(* Logix 5000 AddOnInstructionDefinition export Banner_QS18E_Param_v3; software revision 30.00 *)

TYPE Banner_IOL_Port_v2 :   // UDT that has all of the data items necessary to communicate with a specific Port on a IO-Link Master
STRUCT
   Port_Controlled : INT;   // Each bit represents a port on an IO-Link Master. Set to 1 to tell AOI to control that port.
   Port_Activate : INT;   // Each bit represents a port on an IO-Link Master. When ON that port will process any commands in queue.
   Port_Read : INT;   // Each bit represents a port on an IO-Link Master. Used to determine when device AOI has requested a Read command.
   Port_Write : INT;   // Each bit represents a port on an IO-Link Master. Used to determine when device AOI has requested a Write command.
   Port_RW_Complete : INT;   // Each bit represents a port on an IO-Link Master. Tells device AOI that Read or Write request has been completed.
   Port_Device_Read : INT;
   Data_Transfer : SINT[70];   // Array to transfer data from IO-Master to device AOIs.
END_STRUCT
END_TYPE

TYPE Banner_QS18E_1 :   // Parameters for D, DV, LP, CV, and FP type sensors.
STRUCT
   Response_Speed : SINT;   // 0 = High Speed, 1 = Standard, 2 = Robust.
   Polarity_of_Pins_2_and_4 : SINT;   // 0 = Push Pull, 1 = PNP, 2 = NPN.
   Pin_2_Config : SINT;   // 0 = Deactivated, 1 = Pin 2 Emitter Enable, 2 = Pin 2 Emitter Disable, 3 = Remote Input, 4 = Detection Output, 5 = Complimentary Output, 6 = Normally Closed Health, 7 = Normally Open Health, 8 = Normally Closed Marginal, 9 = Normally Open Marginal.
   Process_Data_Input_Config : SINT;   // 0 = 5 and Signal, 1 = 5 and Count, 2 = 5 and Duration, 3 = 5 and Events per Minute.
   Marginal_Mode : SINT;   // 0 = Marginal Disabled, 1 = Marginal Auto, 2 = Marginal User.
   User_Marginal_Light : INT;   // 0 to 1000. User defined threshold.
   User_Marginal_Dark : INT;   // 0 to 1000. User defined threshold.
   LED_Power : SINT;   // 0 = Auto, 1 = Min Power, 2 = Power 2, 3 = Power 3, 4 = Power 4, 5 = Power 5, 6 = Max Power.
END_STRUCT
END_TYPE

TYPE Banner_QS18E_2 :   // Parameters for EV and E type sensors
STRUCT
   Polarity_of_Pins_2_and_4 : SINT;   // 0 = Push Pull, 1 = PNP, 2 = NPN.
   Pin_2_Config : SINT;   // 0 = Deactivated, 1 = Pin 2 Emitter Enable, 2 = Pin 2 Emitter Disable, 3 = Remote Input, 4 = Detection Output, 5 = Complimentary Output, 6 = Normally Closed Health, 7 = Normally Open Health, 8 = Normally Closed Marginal, 9 = Normally Open Marginal.
   Frequency_Selection : SINT;   // 0 = High Speed, 1 = A, 2 = B, 3 = C.
   Power_Level : SINT;   // 0 to 5. Example: 5 = Power Level 5.
   Pushbutton_Lockout : SINT;   // 0 = Unlocked, 1 = Locked.
END_STRUCT
END_TYPE

TYPE Banner_QS18E_3 :   // Parameters for RV and R type sensors
STRUCT
   Polarity_of_Pins_2_and_4 : SINT;   // 0 = Push Pull, 1 = PNP, 2 = NPN.
   Pin_2_Config : SINT;   // 0 = Deactivated, 1 = Pin 2 Emitter Enable, 2 = Pin 2 Emitter Disable, 3 = Remote Input, 4 = Detection Output, 5 = Complimentary Output, 6 = Normally Closed Health, 7 = Normally Open Health, 8 = Normally Closed Marginal, 9 = Normally Open Marginal.
   Process_Data_Input_Config : SINT;   // 0 = 5 and Signal, 1 = 5 and Count, 2 = 5 and Duration, 3 = 5 and Events per Minute.
   Marginal_Mode : SINT;   // 0 = Marginal Disabled, 1 = Marginal Auto, 2 = Marginal User.
   User_Marginal_Light : INT;   // 0 to 1000. User defined threshold.
   User_Marginal_Dark : INT;   // 0 to 1000. User defined threshold.
   Frequency_Selection : SINT;   // 0 = High Speed, 1 = A, 2 = B, 3 = C.
   IOL_Filter_Time : INT;   // Time in ms to average IOL process data measurement between updates.
   Gain : SINT;   // 0 = Auto - Teach, 1 = Auto - Run, 2 = Low Gain, 3 = Mid Gain, 4 = High Gain.
   Pushbutton_Lockout : SINT;   // 0 = Unlocked, 1 = Locked.
END_STRUCT
END_TYPE

TYPE Banner_QS18E_RD_v3 :   // UDT that stores the Write Data for a QS18E.
STRUCT
   Master_Cycle_Time : INT;
   Min_Cycle_Time : INT;
   M_Sequence_Capability : INT;
   IO_Link_Version_ID : INT;
   Process_Data_Input_Length : INT;
   Process_Data_Output_Length : INT;
   Combined_Vendor_ID : DINT;   // IO-Link Vendor ID
   Vendor_ID1 : INT;
   Vendor_ID2 : INT;
   Combined_Device_ID : DINT;   // IO-Link Device ID
   Device_ID1 : INT;
   Device_ID2 : INT;
   Device_ID3 : INT;
   Serial_Number : STRING;
   All_Time_Run_Time : DINT;   // Read only counter that tracks the total time sensor has been running since manufacture. Value in Hours.
   Quality_of_Health : INT;
   Normalized_Signal_Strength : INT;
   Quality_of_Teach : INT;
   Health_Lower_Limit : INT;
   Health_Upper_Limit : INT;
   SP2_Lower_Sensing_Threshold : INT;
   SP2_Upper_Sensing_Threshold : INT;
   SP1_Lower_Sensing_Threshold : INT;
   SP1_Upper_Sensing_Threshold : INT;
   Sensor_Operationl_Mode : INT;
   Output_Event_Count : DINT;
   Output_Event_Duration : DINT;
   Output_Event_Frequency : DINT;
   Active_Margninal_Light_Threshold : DINT;
   Active_Marginal_Dark_Threshold : DINT;
   Sigal : DINT;   // Only available for Sensor Type 3. Raw ADC Signal value.
END_STRUCT
END_TYPE

TYPE Banner_QS18E_v3 :   // All of the parameters for a QS18E.
STRUCT
   Initial_Global_Read : BOOL;   // Determines if all of the IO-Link data has been read into the PLC yet
   Command : INT;   // Value placed in here will activate a read or write to a specifc IO-Link Index
   Read_Data : Banner_QS18E_RD_v3;   // Read Only Data
   Write_Data : Banner_QS18E_WD_v3;   // Write Data
   Archive : Banner_QS18E_WD_v3;   // Archive Data
   Reset : BOOL;   // Resets AOI. This will force a complete parameter read of the sensor.
END_STRUCT
END_TYPE

TYPE Banner_QS18E_WD_v3 :   // UDT that stores the Write Data for a QS18E.
STRUCT
   System_Command : INT;   // See IODD file for list of commands that can be activated via the System Command interface
   Parameter_Access_Lock : SINT;   // Write access to all parameters is prohibited while value is 1. Only this parameter can be adjusted when value is 1.
   Data_Storage_Lock : SINT;   // Automatic data storage is disabled when this value is equal to 1. Read access is not affected.
   Local_Parameterization_Lock : SINT;   // Parameterization via local control elements on device is disabled.
   Local_User_Interface_Lock : SINT;   // Operation of local user interface is disabled.
   BDC1_Swithpoint_Logic : INT;   // 0 = Light Operate, 1 = Dark Operate
   BDC1_BDC_Mode : INT;   // 1 = 1-Pt BGS, 128 = 2-Pt, 129 = Dynamic, 130 = Window or FGS, 131 = Dual
   BDC1_Hysteresis : DINT;   // Should always be 0
   Marginal_Signal_Delay : DINT;   // 0 to 60000. Millisecond value
   User_Health_Setting : INT;   // 0 to 90
   Offset_Percent : INT;   // 0 = Min, 1 = 10%, 2 = 15%, 3 = 20%, 4 = 25%, 5 = 30%, 6 = 40%, 7 = 50%, 8 = 100%, 9 = 200%.
   Auto_Compensaton : INT;   // 0=Disabled, 1=Enabled
   Delay_Timer_2 : DINT;   // 0 to 90000 ms
   Delay_Timer_1 : DINT;   // 0 to 90000 ms
   Delay_Mode : INT;   // 0=Disabled, 1=On Off Delay, 2=On One Shot, 3=Off One Shot
   Resettable_Run_Time : DINT;
   Type_1_Data : Banner_QS18E_1;   // Data for a D, DV, Lp, VC, or FP QS18E type sensor.
   Type_2_Data : Banner_QS18E_2;   // Data for a E or EV QS18E type sensor.
   Type_3_Data : Banner_QS18E_3;   // Data for a R or RV QS18E type sensor.
   All_Time_Run_Time_Event_Time : DINT;
   Resettable_Run_Time_Event_Time : DINT;
END_STRUCT
END_TYPE

ADD_ON_INSTRUCTION Banner_QS18E_Param_v3   (* revision 3.0, vendor Banner Engineering *)
// AOI to read and write parameter data to an IO-Link QS18E.
// Revision note:
// Updated for QS18 Emitter and Receiver.
VAR_IN_OUT
   QS18E : Banner_QS18E_v3; {required}
   Port_Data : Banner_IOL_Port_v2; {required}
END_VAR
VAR_INPUT
   Port : DINT; {required}
   Sensor_Type : DINT; {required}   // 1 = D, DV, LP, CV, & FP models, 2 = EV or E models, 3 = RV or R models.
END_VAR
VAR
   Local_Control : DINT; {access None}
   Global_Read_Command_Value : INT; {access None}
   Global_Write_Command_Value : INT; {access None}
   Command_Being_Processed : BOOL; {access None}
   Update_Archive : BOOL; {access None}
   Index_Write_Inprocess : INT; {access None}
   Index_Write_Control : INT; {access None}
   Inprocess_Index : DINT; {access None}
END_VAR

ROUTINE Logic   (* ladder *)
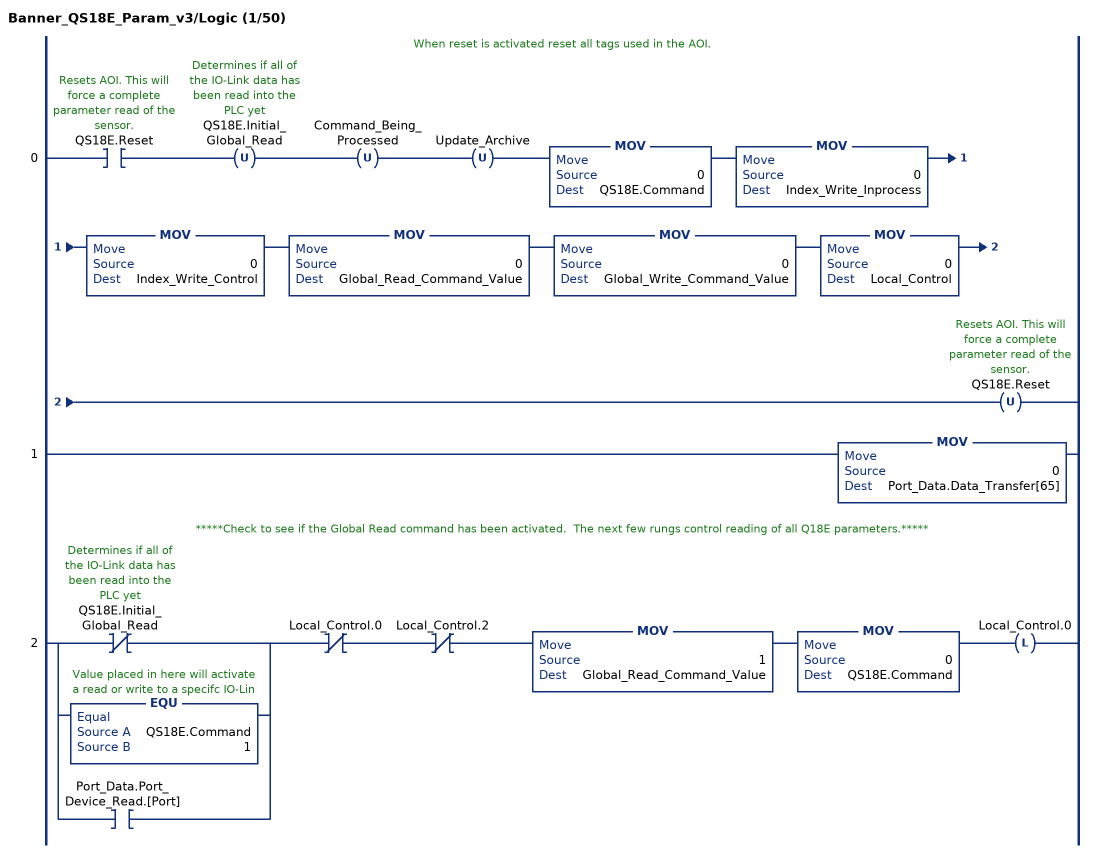
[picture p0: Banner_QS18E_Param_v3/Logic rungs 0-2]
   // When reset is activated reset all tags used in the AOI.
   0: XIC(QS18E.Reset)OTU(QS18E.Initial_Global_Read)OTU(Command_Being_Processed)OTU(Update_Archive)MOV(0,QS18E.Command)MOV(0,Index_Write_Inprocess)MOV(0,Index_Write_Control)MOV(0,Global_Read_Command_Value)MOV(0,Global_Write_Command_Value)MOV(0,Local_Control)OTU(QS18E.Reset);
   1: MOV(0,Port_Data.Data_Transfer[65]);
   // *****Check to see if the Global Read command has been activated.  The next few rungs control reading of all Q18E parameters.*****
   2: [XIO(QS18E.Initial_Global_Read) ,EQU(QS18E.Command,1) ,XIC(Port_Data.Port_Device_Read.[Port]) ]XIO(Local_Control.0)XIO(Local_Control.2)MOV(1,Global_Read_Command_Value)MOV(0,QS18E.Command)OTL(Local_Control.0);
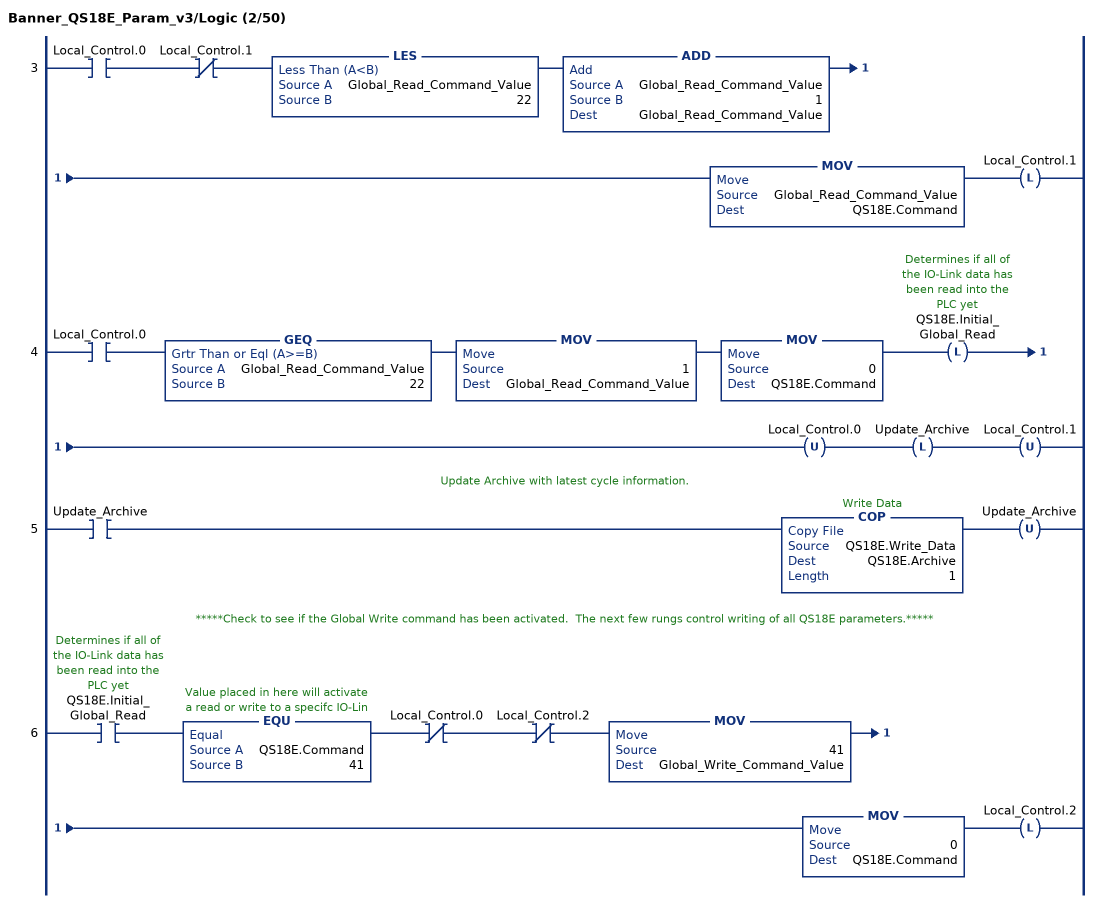
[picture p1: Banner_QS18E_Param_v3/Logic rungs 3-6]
   3: XIC(Local_Control.0)XIO(Local_Control.1)LES(Global_Read_Command_Value,22)ADD(Global_Read_Command_Value,1,Global_Read_Command_Value)MOV(Global_Read_Command_Value,QS18E.Command)OTL(Local_Control.1);
   4: XIC(Local_Control.0)GEQ(Global_Read_Command_Value,22)MOV(1,Global_Read_Command_Value)MOV(0,QS18E.Command)OTL(QS18E.Initial_Global_Read)OTU(Local_Control.0)OTL(Update_Archive)OTU(Local_Control.1);
   // Update Archive with latest cycle information.
   5: XIC(Update_Archive)COP(QS18E.Write_Data,QS18E.Archive,1)OTU(Update_Archive);
   // *****Check to see if the Global Write command has been activated.  The next few rungs control writing of all QS18E parameters.*****
   6: XIC(QS18E.Initial_Global_Read)EQU(QS18E.Command,41)XIO(Local_Control.0)XIO(Local_Control.2)MOV(41,Global_Write_Command_Value)MOV(0,QS18E.Command)OTL(Local_Control.2);
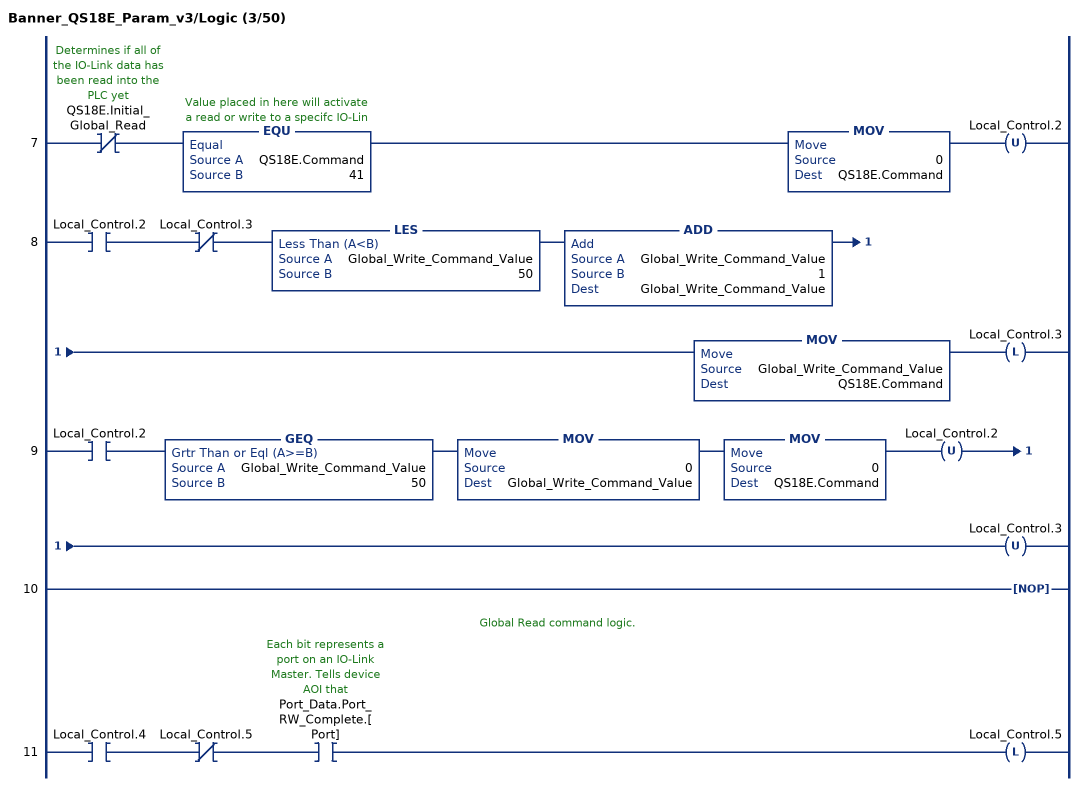
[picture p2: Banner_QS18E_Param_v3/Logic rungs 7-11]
   7: XIO(QS18E.Initial_Global_Read)EQU(QS18E.Command,41)MOV(0,QS18E.Command)OTU(Local_Control.2);
   8: XIC(Local_Control.2)XIO(Local_Control.3)LES(Global_Write_Command_Value,50)ADD(Global_Write_Command_Value,1,Global_Write_Command_Value)MOV(Global_Write_Command_Value,QS18E.Command)OTL(Local_Control.3);
   9: XIC(Local_Control.2)GEQ(Global_Write_Command_Value,50)MOV(0,Global_Write_Command_Value)MOV(0,QS18E.Command)OTU(Local_Control.2)OTU(Local_Control.3);
   10: NOP();
   // Global Read command logic.
   11: XIC(Local_Control.4)XIO(Local_Control.5)XIC(Port_Data.Port_RW_Complete.[Port])OTL(Local_Control.5);
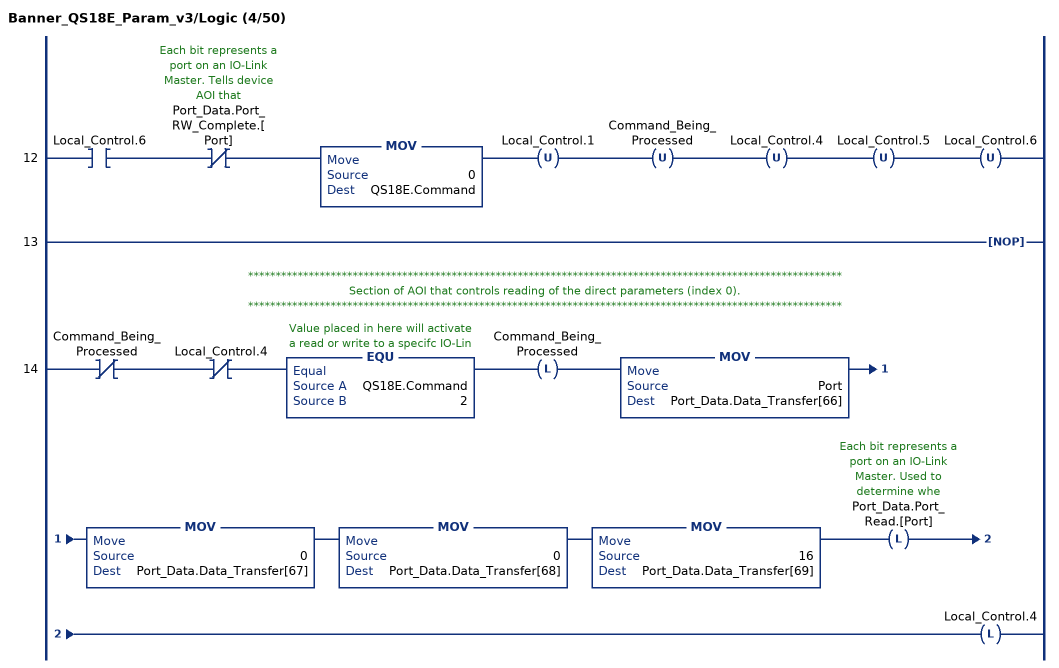
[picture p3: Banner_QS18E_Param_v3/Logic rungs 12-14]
   12: XIC(Local_Control.6)XIO(Port_Data.Port_RW_Complete.[Port])MOV(0,QS18E.Command)OTU(Local_Control.1)OTU(Command_Being_Processed)OTU(Local_Control.4)OTU(Local_Control.5)OTU(Local_Control.6);
   13: NOP();
   // ************************************************************************************************************
   // Section of AOI that controls reading of the direct parameters (index 0).
   // ************************************************************************************************************
   14: XIO(Command_Being_Processed)XIO(Local_Control.4)EQU(QS18E.Command,2)OTL(Command_Being_Processed)MOV(Port,Port_Data.Data_Transfer[66])MOV(0,Port_Data.Data_Transfer[67])MOV(0,Port_Data.Data_Transfer[68])MOV(16,Port_Data.Data_Transfer[69])OTL(Port_Data.Port_Read.[Port])OTL(Local_Control.4);
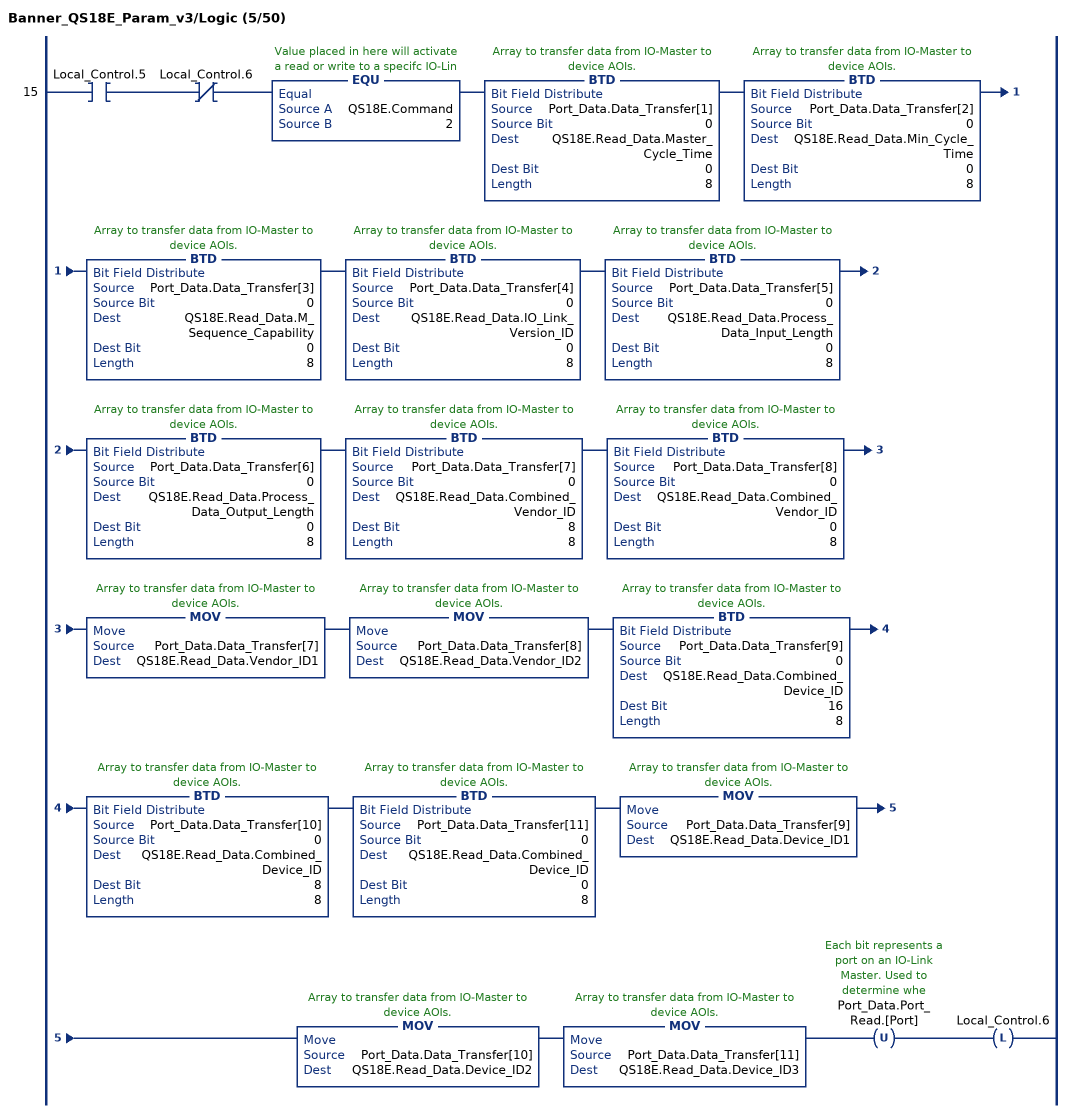
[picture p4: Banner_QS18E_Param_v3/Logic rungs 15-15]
   15: XIC(Local_Control.5)XIO(Local_Control.6)EQU(QS18E.Command,2)BTD(Port_Data.Data_Transfer[1],0,QS18E.Read_Data.Master_Cycle_Time,0,8)BTD(Port_Data.Data_Transfer[2],0,QS18E.Read_Data.Min_Cycle_Time,0,8)BTD(Port_Data.Data_Transfer[3],0,QS18E.Read_Data.M_Sequence_Capability,0,8)BTD(Port_Data.Data_Transfer[4],0,QS18E.Read_Data.IO_Link_Version_ID,0,8)BTD(Port_Data.Data_Transfer[5],0,QS18E.Read_Data.Process_Data_Input_Length,0,8)BTD(Port_Data.Data_Transfer[6],0,QS18E.Read_Data.Process_Data_Output_Length,0,8)BTD(Port_Data.Data_Transfer[7],0,QS18E.Read_Data.Combined_Vendor_ID,8,8)BTD(Port_Data.Data_Transfer[8],0,QS18E.Read_Data.Combined_Vendor_ID,0,8)MOV(Port_Data.Data_Transfer[7],QS18E.Read_Data.Vendor_ID1)MOV(Port_Data.Data_Transfer[8],QS18E.Read_Data.Vendor_ID2)BTD(Port_Data.Data_Transfer[9],0,QS18E.Read_Data.Combined_Device_ID,16,8)BTD(Port_Data.Data_Transfer[10],0,QS18E.Read_Data.Combined_Device_ID,8,8)BTD(Port_Data.Data_Transfer[11],0,QS18E.Read_Data.Combined_Device_ID,0,8)MOV(Port_Data.Data_Transfer[9],QS18E.Read_Data.Device_ID1)MOV(Port_Data.Data_Transfer[10],QS18E.Read_Data.Device_ID2)MOV(Port_Data.Data_Transfer[11],QS18E.Read_Data.Device_ID3)OTU(Port_Data.Port_Read.[Port])OTL(Local_Control.6);
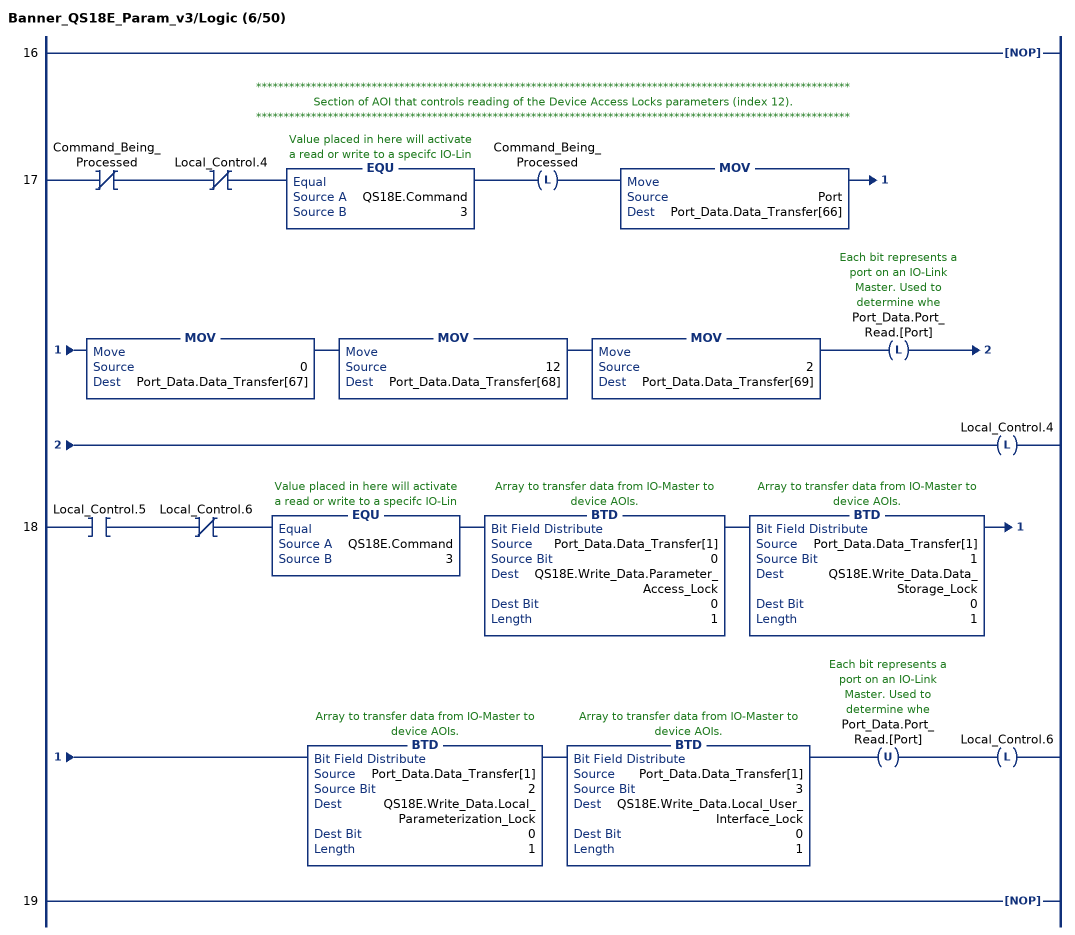
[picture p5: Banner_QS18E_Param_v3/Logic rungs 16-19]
   16: NOP();
   // ************************************************************************************************************
   // Section of AOI that controls reading of the Device Access Locks parameters (index 12).
   // ************************************************************************************************************
   17: XIO(Command_Being_Processed)XIO(Local_Control.4)EQU(QS18E.Command,3)OTL(Command_Being_Processed)MOV(Port,Port_Data.Data_Transfer[66])MOV(0,Port_Data.Data_Transfer[67])MOV(12,Port_Data.Data_Transfer[68])MOV(2,Port_Data.Data_Transfer[69])OTL(Port_Data.Port_Read.[Port])OTL(Local_Control.4);
   18: XIC(Local_Control.5)XIO(Local_Control.6)EQU(QS18E.Command,3)BTD(Port_Data.Data_Transfer[1],0,QS18E.Write_Data.Parameter_Access_Lock,0,1)BTD(Port_Data.Data_Transfer[1],1,QS18E.Write_Data.Data_Storage_Lock,0,1)BTD(Port_Data.Data_Transfer[1],2,QS18E.Write_Data.Local_Parameterization_Lock,0,1)BTD(Port_Data.Data_Transfer[1],3,QS18E.Write_Data.Local_User_Interface_Lock,0,1)OTU(Port_Data.Port_Read.[Port])OTL(Local_Control.6);
   19: NOP();
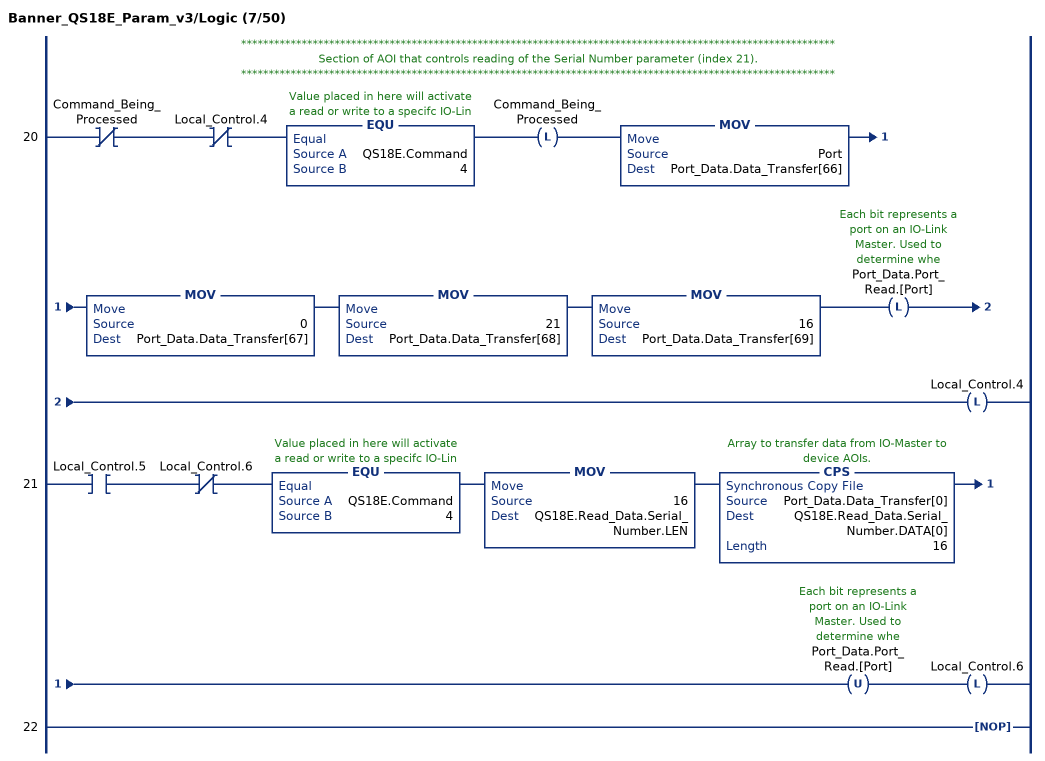
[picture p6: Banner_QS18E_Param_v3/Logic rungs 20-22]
   // ************************************************************************************************************
   // Section of AOI that controls reading of the Serial Number parameter (index 21).
   // ************************************************************************************************************
   20: XIO(Command_Being_Processed)XIO(Local_Control.4)EQU(QS18E.Command,4)OTL(Command_Being_Processed)MOV(Port,Port_Data.Data_Transfer[66])MOV(0,Port_Data.Data_Transfer[67])MOV(21,Port_Data.Data_Transfer[68])MOV(16,Port_Data.Data_Transfer[69])OTL(Port_Data.Port_Read.[Port])OTL(Local_Control.4);
   21: XIC(Local_Control.5)XIO(Local_Control.6)EQU(QS18E.Command,4)MOV(16,QS18E.Read_Data.Serial_Number.LEN)CPS(Port_Data.Data_Transfer[0],QS18E.Read_Data.Serial_Number.DATA[0],16)OTU(Port_Data.Port_Read.[Port])OTL(Local_Control.6);
   22: NOP();
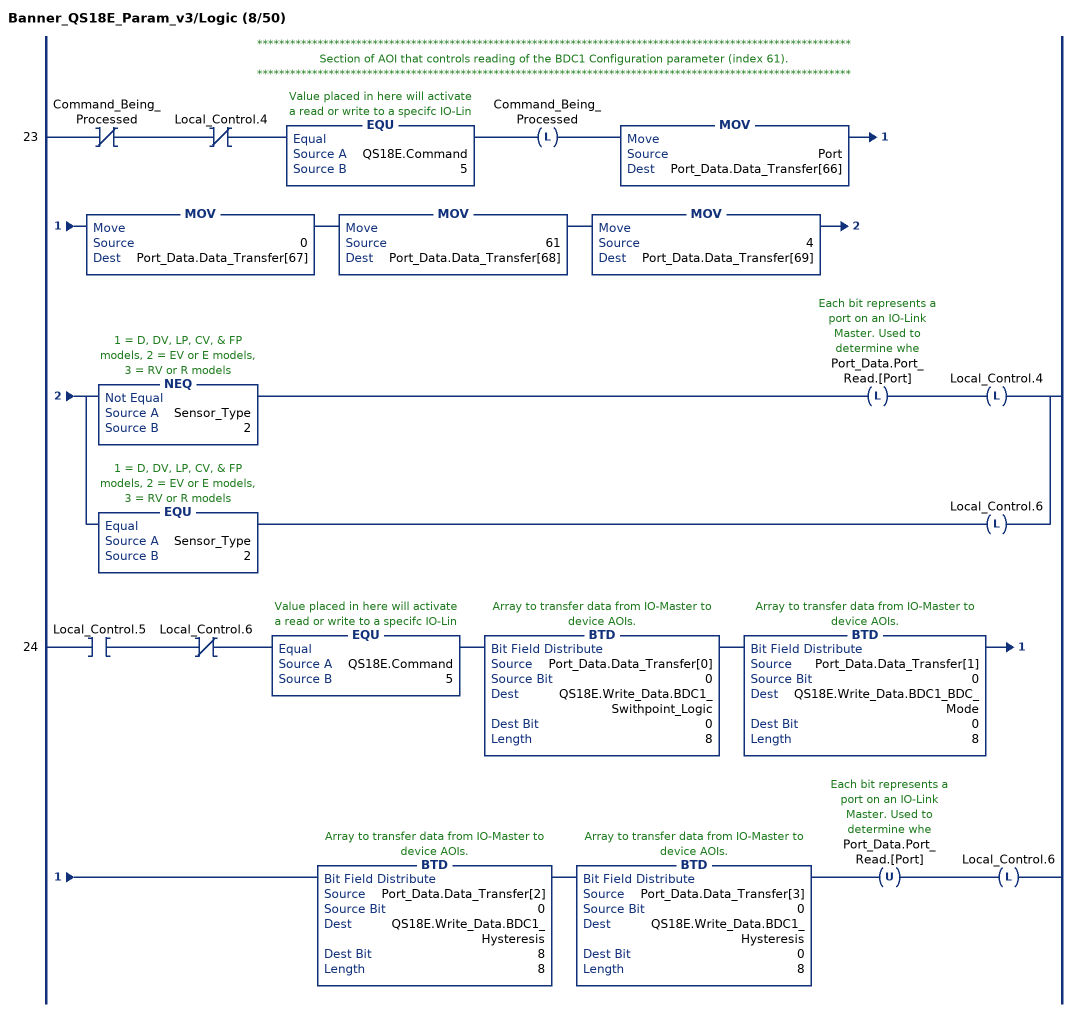
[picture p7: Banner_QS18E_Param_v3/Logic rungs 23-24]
   // ************************************************************************************************************
   // Section of AOI that controls reading of the BDC1 Configuration parameter (index 61).
   // ************************************************************************************************************
   23: XIO(Command_Being_Processed)XIO(Local_Control.4)EQU(QS18E.Command,5)OTL(Command_Being_Processed)MOV(Port,Port_Data.Data_Transfer[66])MOV(0,Port_Data.Data_Transfer[67])MOV(61,Port_Data.Data_Transfer[68])MOV(4,Port_Data.Data_Transfer[69])[NEQ(Sensor_Type,2) OTL(Port_Data.Port_Read.[Port]) OTL(Local_Control.4) ,EQU(Sensor_Type,2) OTL(Local_Control.6) ];
   24: XIC(Local_Control.5)XIO(Local_Control.6)EQU(QS18E.Command,5)BTD(Port_Data.Data_Transfer[0],0,QS18E.Write_Data.BDC1_Swithpoint_Logic,0,8)BTD(Port_Data.Data_Transfer[1],0,QS18E.Write_Data.BDC1_BDC_Mode,0,8)BTD(Port_Data.Data_Transfer[2],0,QS18E.Write_Data.BDC1_Hysteresis,8,8)BTD(Port_Data.Data_Transfer[3],0,QS18E.Write_Data.BDC1_Hysteresis,0,8)OTU(Port_Data.Port_Read.[Port])OTL(Local_Control.6);
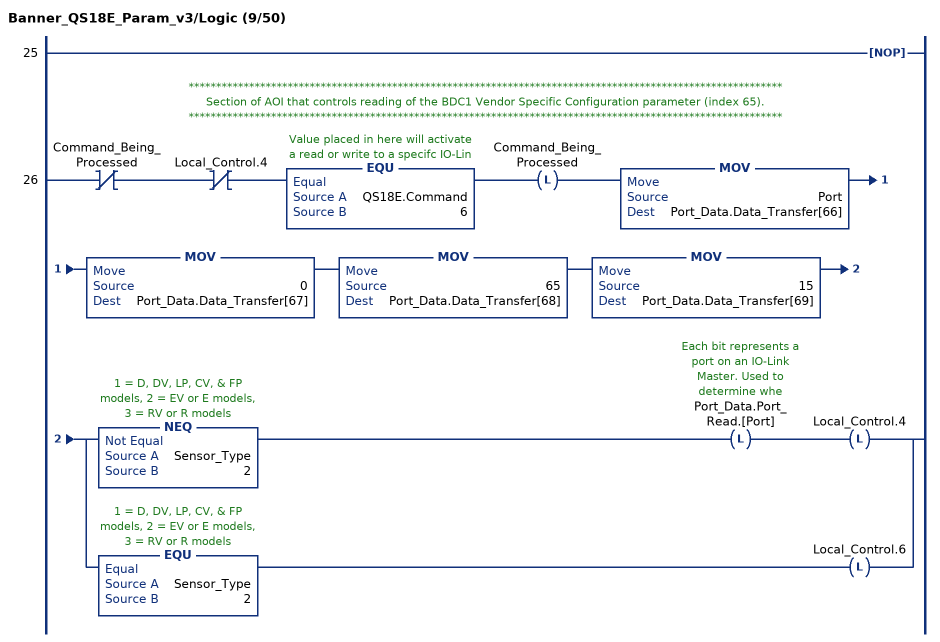
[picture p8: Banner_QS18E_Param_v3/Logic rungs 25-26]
   25: NOP();
   // ************************************************************************************************************
   // Section of AOI that controls reading of the BDC1 Vendor Specific Configuration parameter (index 65).
   // ************************************************************************************************************
   26: XIO(Command_Being_Processed)XIO(Local_Control.4)EQU(QS18E.Command,6)OTL(Command_Being_Processed)MOV(Port,Port_Data.Data_Transfer[66])MOV(0,Port_Data.Data_Transfer[67])MOV(65,Port_Data.Data_Transfer[68])MOV(15,Port_Data.Data_Transfer[69])[NEQ(Sensor_Type,2) OTL(Port_Data.Port_Read.[Port]) OTL(Local_Control.4) ,EQU(Sensor_Type,2) OTL(Local_Control.6) ];
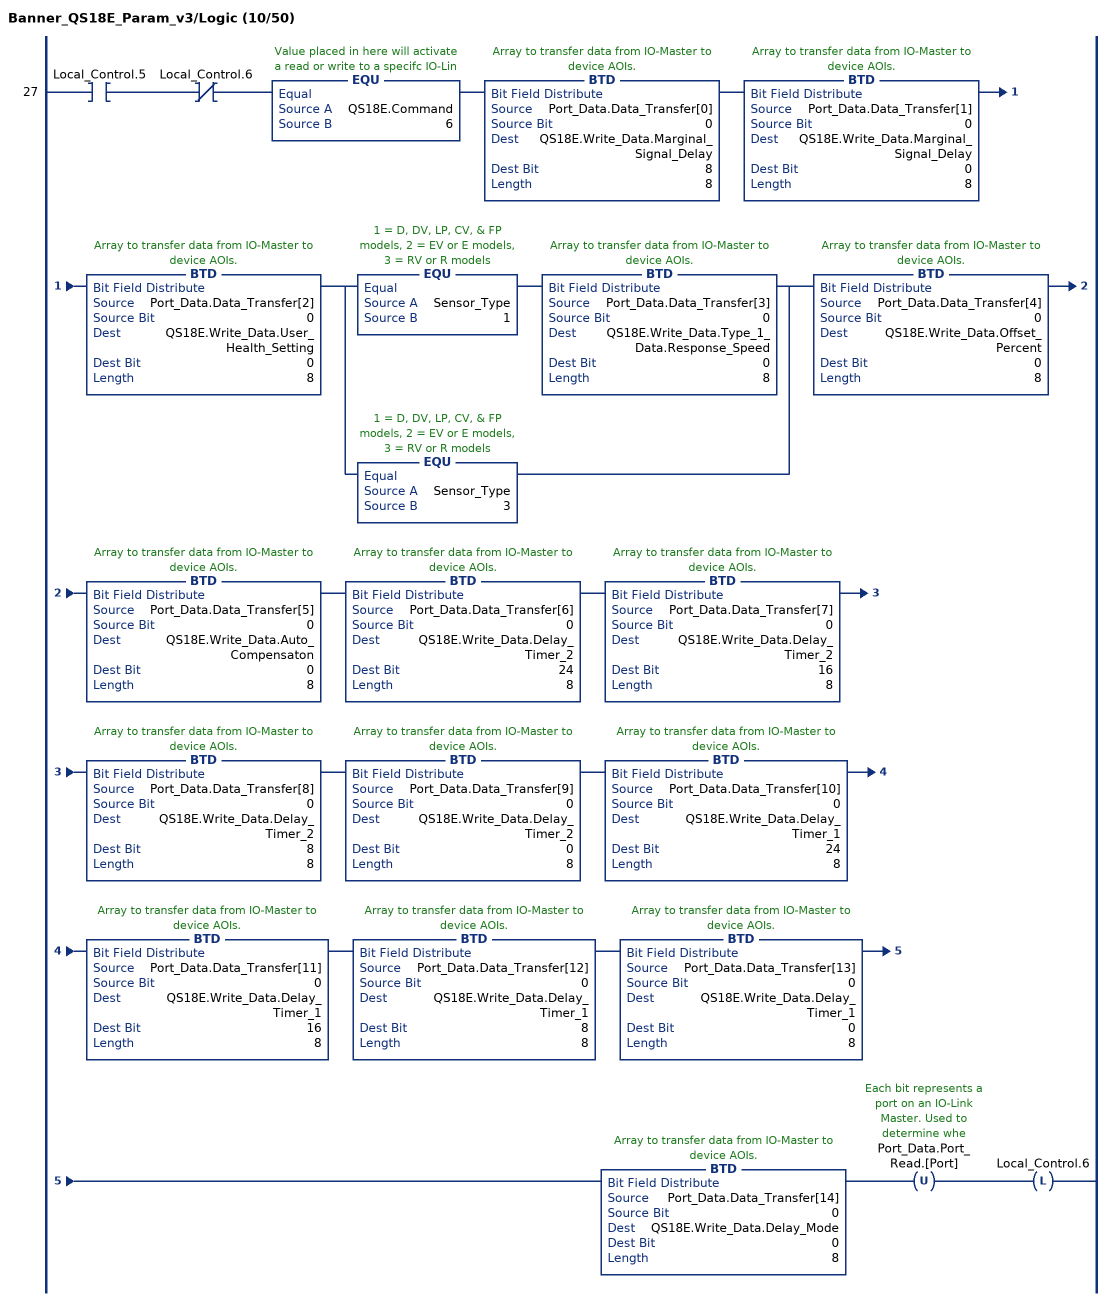
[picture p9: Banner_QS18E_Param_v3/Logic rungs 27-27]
   27: XIC(Local_Control.5)XIO(Local_Control.6)EQU(QS18E.Command,6)BTD(Port_Data.Data_Transfer[0],0,QS18E.Write_Data.Marginal_Signal_Delay,8,8)BTD(Port_Data.Data_Transfer[1],0,QS18E.Write_Data.Marginal_Signal_Delay,0,8)BTD(Port_Data.Data_Transfer[2],0,QS18E.Write_Data.User_Health_Setting,0,8)[EQU(Sensor_Type,1) BTD(Port_Data.Data_Transfer[3],0,QS18E.Write_Data.Type_1_Data.Response_Speed,0,8) ,EQU(Sensor_Type,3) ]BTD(Port_Data.Data_Transfer[4],0,QS18E.Write_Data.Offset_Percent,0,8)BTD(Port_Data.Data_Transfer[5],0,QS18E.Write_Data.Auto_Compensaton,0,8)BTD(Port_Data.Data_Transfer[6],0,QS18E.Write_Data.Delay_Timer_2,24,8)BTD(Port_Data.Data_Transfer[7],0,QS18E.Write_Data.Delay_Timer_2,16,8)BTD(Port_Data.Data_Transfer[8],0,QS18E.Write_Data.Delay_Timer_2,8,8)BTD(Port_Data.Data_Transfer[9],0,QS18E.Write_Data.Delay_Timer_2,0,8)BTD(Port_Data.Data_Transfer[10],0,QS18E.Write_Data.Delay_Timer_1,24,8)BTD(Port_Data.Data_Transfer[11],0,QS18E.Write_Data.Delay_Timer_1,16,8)BTD(Port_Data.Data_Transfer[12],0,QS18E.Write_Data.Delay_Timer_1,8,8)BTD(Port_Data.Data_Transfer[13],0,QS18E.Write_Data.Delay_Timer_1,0,8)BTD(Port_Data.Data_Transfer[14],0,QS18E.Write_Data.Delay_Mode,0,8)OTU(Port_Data.Port_Read.[Port])OTL(Local_Control.6);
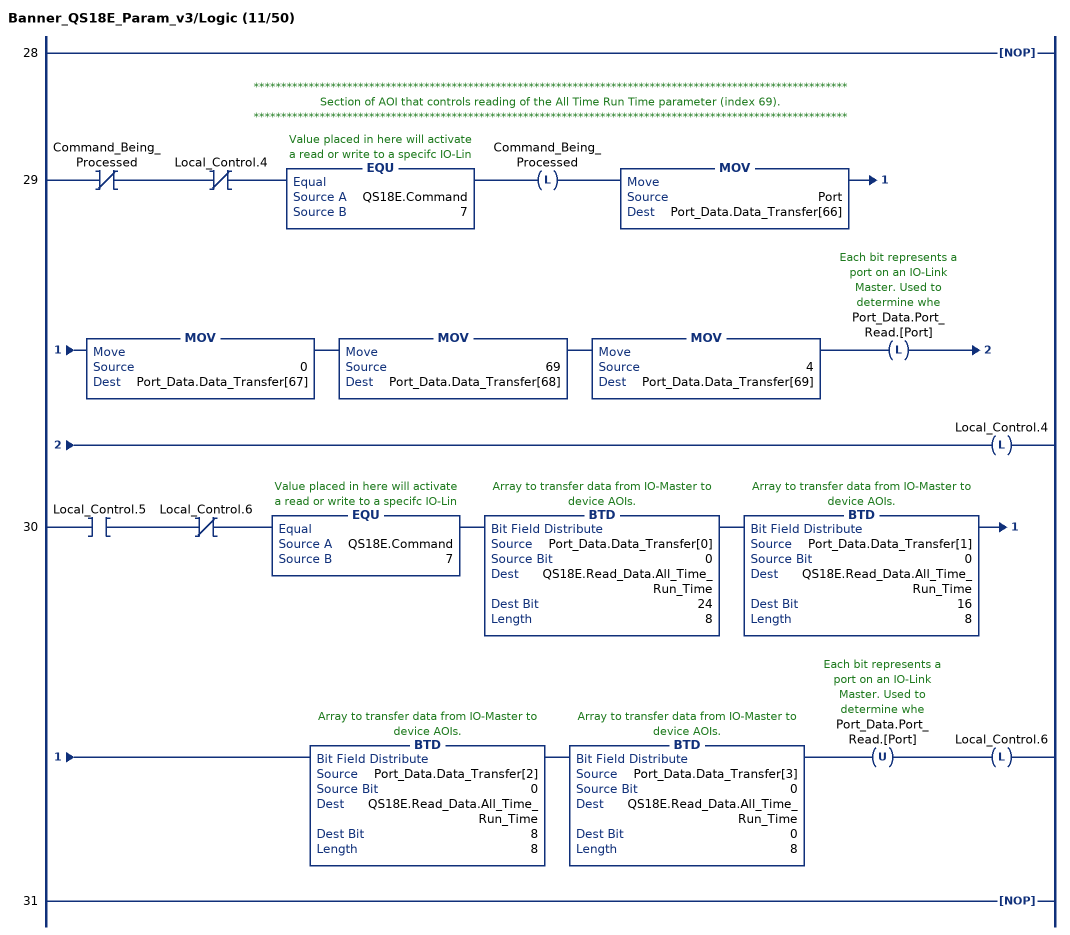
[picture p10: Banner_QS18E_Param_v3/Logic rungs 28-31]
   28: NOP();
   // ************************************************************************************************************
   // Section of AOI that controls reading of the All Time Run Time parameter (index 69).
   // ************************************************************************************************************
   29: XIO(Command_Being_Processed)XIO(Local_Control.4)EQU(QS18E.Command,7)OTL(Command_Being_Processed)MOV(Port,Port_Data.Data_Transfer[66])MOV(0,Port_Data.Data_Transfer[67])MOV(69,Port_Data.Data_Transfer[68])MOV(4,Port_Data.Data_Transfer[69])OTL(Port_Data.Port_Read.[Port])OTL(Local_Control.4);
   30: XIC(Local_Control.5)XIO(Local_Control.6)EQU(QS18E.Command,7)BTD(Port_Data.Data_Transfer[0],0,QS18E.Read_Data.All_Time_Run_Time,24,8)BTD(Port_Data.Data_Transfer[1],0,QS18E.Read_Data.All_Time_Run_Time,16,8)BTD(Port_Data.Data_Transfer[2],0,QS18E.Read_Data.All_Time_Run_Time,8,8)BTD(Port_Data.Data_Transfer[3],0,QS18E.Read_Data.All_Time_Run_Time,0,8)OTU(Port_Data.Port_Read.[Port])OTL(Local_Control.6);
   31: NOP();
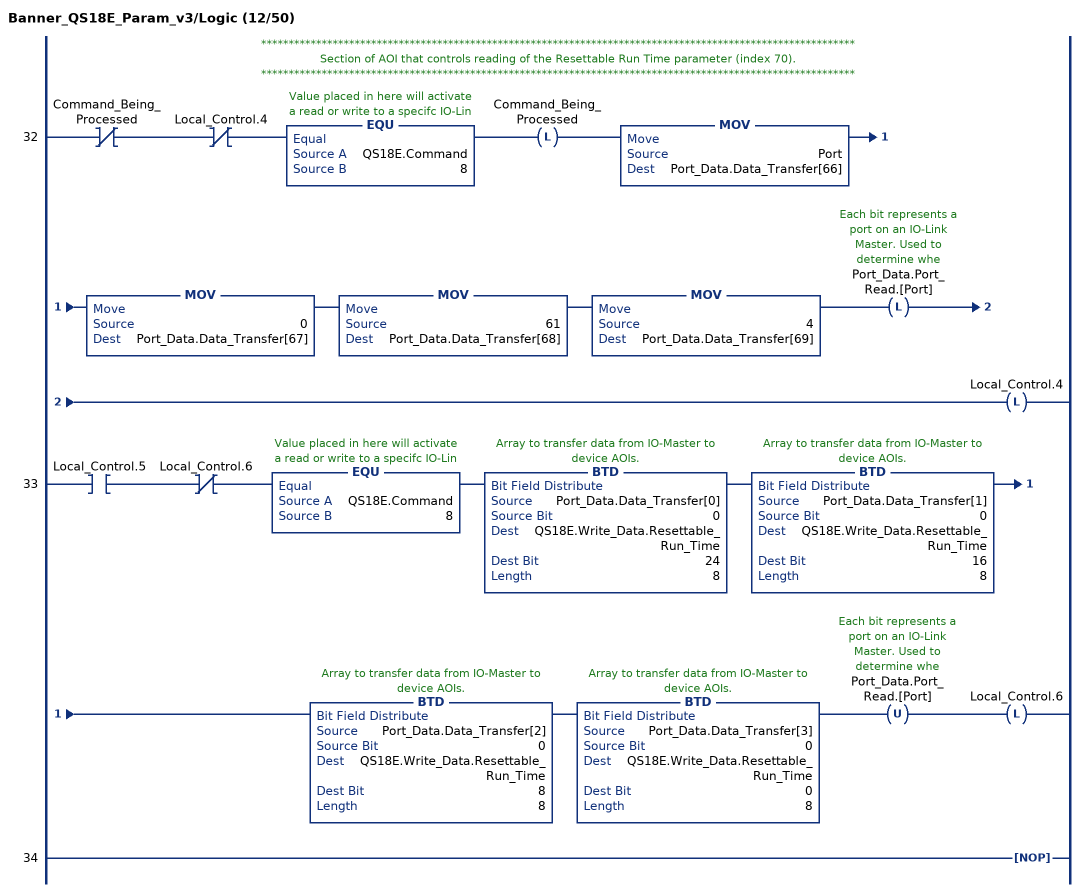
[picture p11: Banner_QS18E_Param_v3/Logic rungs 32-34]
   // ************************************************************************************************************
   // Section of AOI that controls reading of the Resettable Run Time parameter (index 70).
   // ************************************************************************************************************
   32: XIO(Command_Being_Processed)XIO(Local_Control.4)EQU(QS18E.Command,8)OTL(Command_Being_Processed)MOV(Port,Port_Data.Data_Transfer[66])MOV(0,Port_Data.Data_Transfer[67])MOV(61,Port_Data.Data_Transfer[68])MOV(4,Port_Data.Data_Transfer[69])OTL(Port_Data.Port_Read.[Port])OTL(Local_Control.4);
   33: XIC(Local_Control.5)XIO(Local_Control.6)EQU(QS18E.Command,8)BTD(Port_Data.Data_Transfer[0],0,QS18E.Write_Data.Resettable_Run_Time,24,8)BTD(Port_Data.Data_Transfer[1],0,QS18E.Write_Data.Resettable_Run_Time,16,8)BTD(Port_Data.Data_Transfer[2],0,QS18E.Write_Data.Resettable_Run_Time,8,8)BTD(Port_Data.Data_Transfer[3],0,QS18E.Write_Data.Resettable_Run_Time,0,8)OTU(Port_Data.Port_Read.[Port])OTL(Local_Control.6);
   34: NOP();
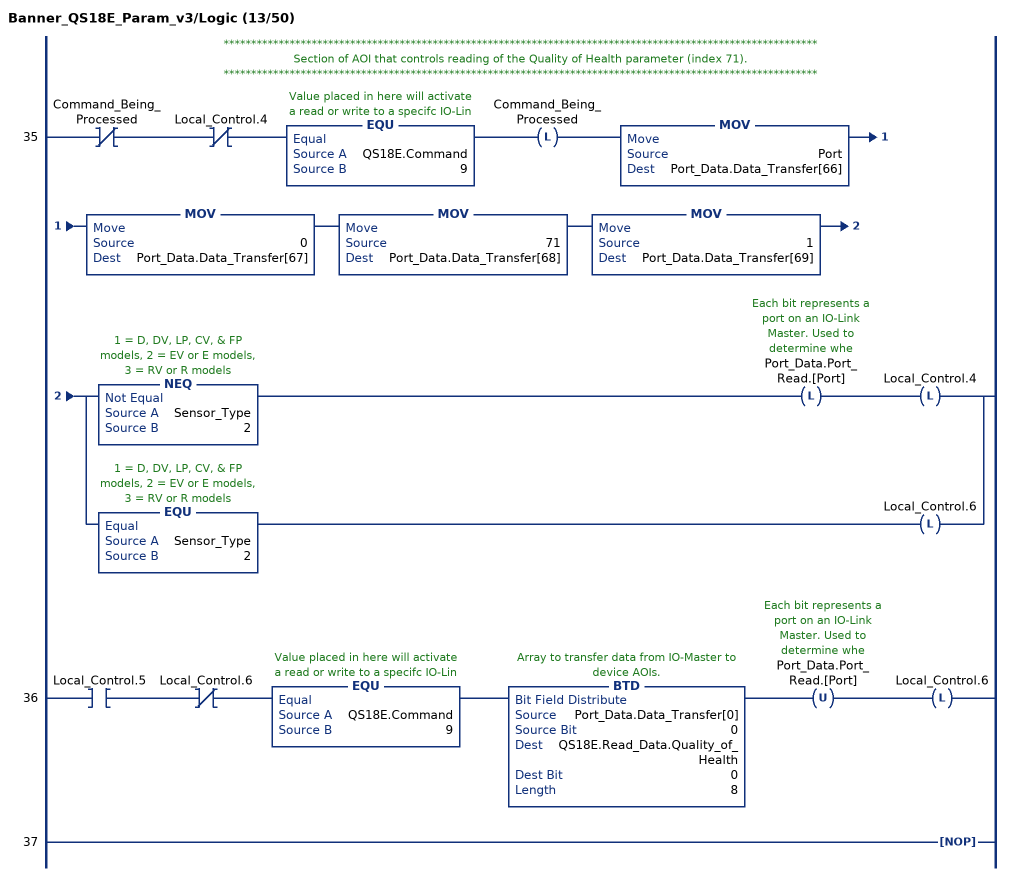
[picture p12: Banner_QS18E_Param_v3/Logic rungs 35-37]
   // ************************************************************************************************************
   // Section of AOI that controls reading of the Quality of Health parameter (index 71).
   // ************************************************************************************************************
   35: XIO(Command_Being_Processed)XIO(Local_Control.4)EQU(QS18E.Command,9)OTL(Command_Being_Processed)MOV(Port,Port_Data.Data_Transfer[66])MOV(0,Port_Data.Data_Transfer[67])MOV(71,Port_Data.Data_Transfer[68])MOV(1,Port_Data.Data_Transfer[69])[NEQ(Sensor_Type,2) OTL(Port_Data.Port_Read.[Port]) OTL(Local_Control.4) ,EQU(Sensor_Type,2) OTL(Local_Control.6) ];
   36: XIC(Local_Control.5)XIO(Local_Control.6)EQU(QS18E.Command,9)BTD(Port_Data.Data_Transfer[0],0,QS18E.Read_Data.Quality_of_Health,0,8)OTU(Port_Data.Port_Read.[Port])OTL(Local_Control.6);
   37: NOP();
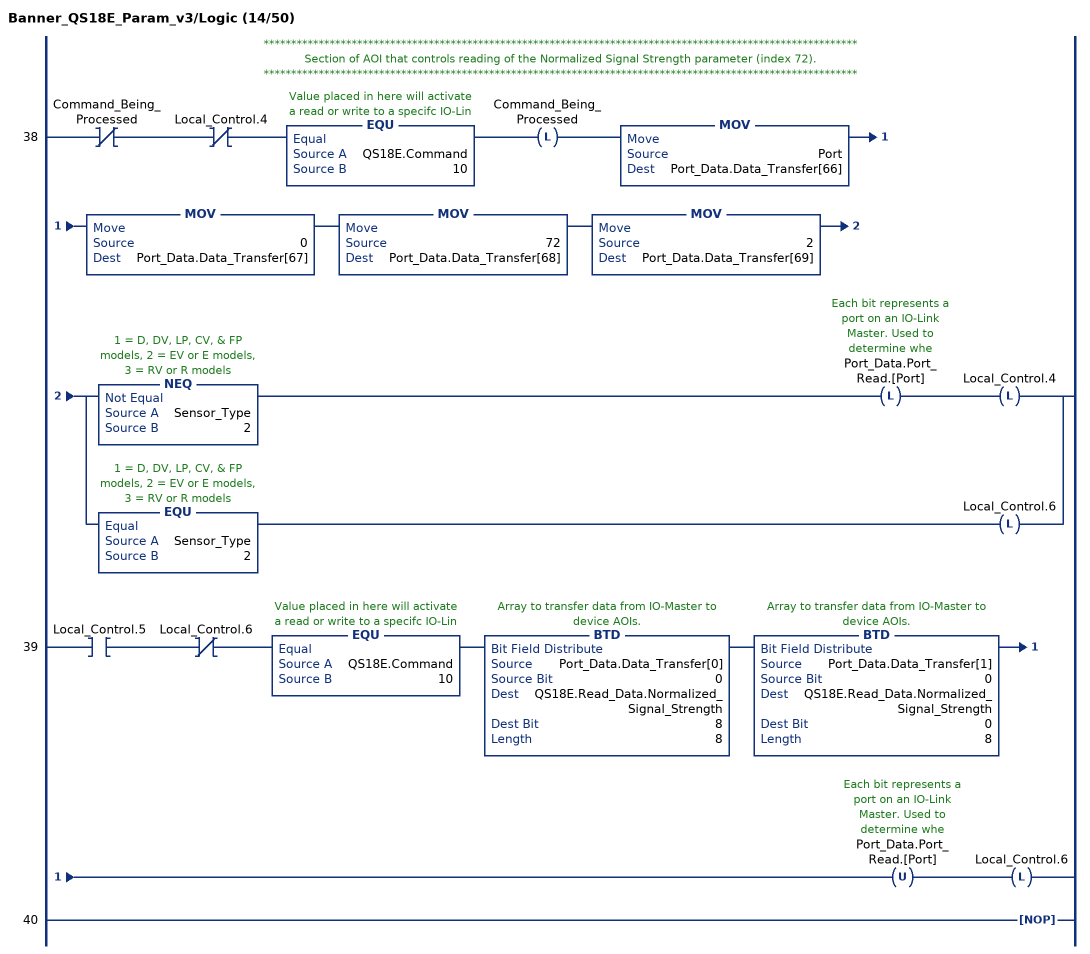
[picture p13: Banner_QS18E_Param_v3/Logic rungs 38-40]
   // ************************************************************************************************************
   // Section of AOI that controls reading of the Normalized Signal Strength parameter (index 72).
   // ************************************************************************************************************
   38: XIO(Command_Being_Processed)XIO(Local_Control.4)EQU(QS18E.Command,10)OTL(Command_Being_Processed)MOV(Port,Port_Data.Data_Transfer[66])MOV(0,Port_Data.Data_Transfer[67])MOV(72,Port_Data.Data_Transfer[68])MOV(2,Port_Data.Data_Transfer[69])[NEQ(Sensor_Type,2) OTL(Port_Data.Port_Read.[Port]) OTL(Local_Control.4) ,EQU(Sensor_Type,2) OTL(Local_Control.6) ];
   39: XIC(Local_Control.5)XIO(Local_Control.6)EQU(QS18E.Command,10)BTD(Port_Data.Data_Transfer[0],0,QS18E.Read_Data.Normalized_Signal_Strength,8,8)BTD(Port_Data.Data_Transfer[1],0,QS18E.Read_Data.Normalized_Signal_Strength,0,8)OTU(Port_Data.Port_Read.[Port])OTL(Local_Control.6);
   40: NOP();
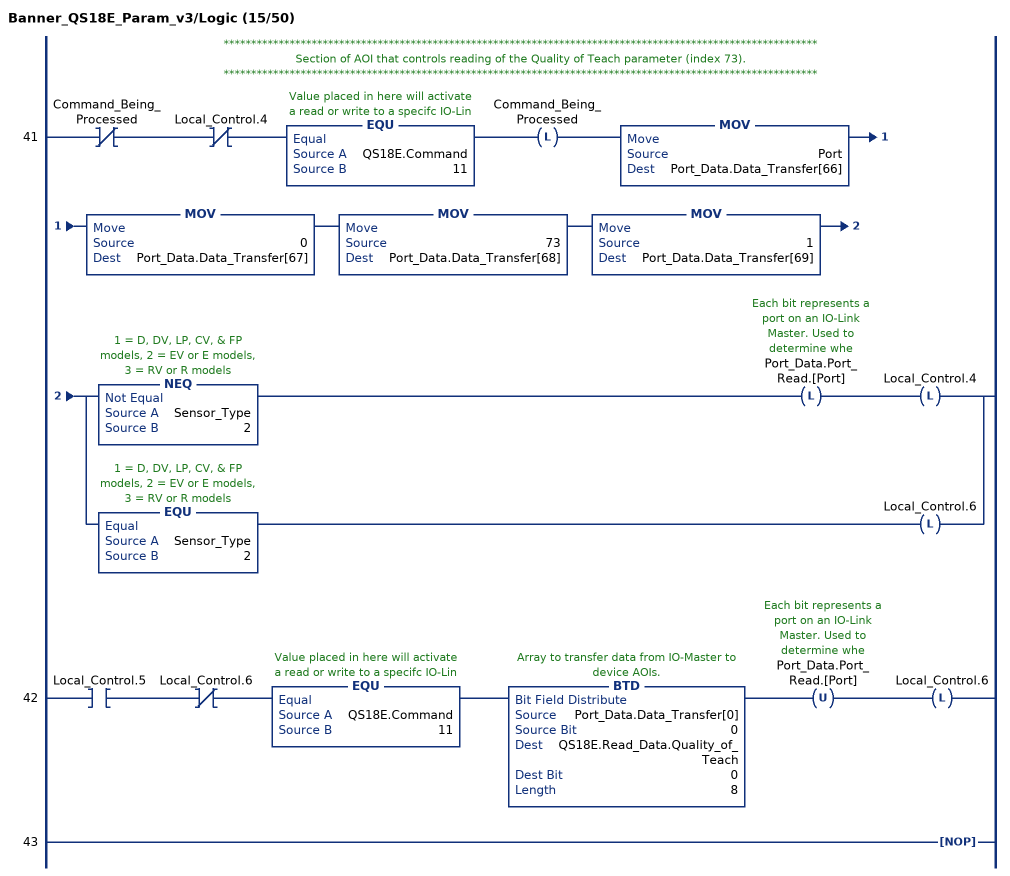
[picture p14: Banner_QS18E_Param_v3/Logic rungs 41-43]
   // ************************************************************************************************************
   // Section of AOI that controls reading of the Quality of Teach parameter (index 73).
   // ************************************************************************************************************
   41: XIO(Command_Being_Processed)XIO(Local_Control.4)EQU(QS18E.Command,11)OTL(Command_Being_Processed)MOV(Port,Port_Data.Data_Transfer[66])MOV(0,Port_Data.Data_Transfer[67])MOV(73,Port_Data.Data_Transfer[68])MOV(1,Port_Data.Data_Transfer[69])[NEQ(Sensor_Type,2) OTL(Port_Data.Port_Read.[Port]) OTL(Local_Control.4) ,EQU(Sensor_Type,2) OTL(Local_Control.6) ];
   42: XIC(Local_Control.5)XIO(Local_Control.6)EQU(QS18E.Command,11)BTD(Port_Data.Data_Transfer[0],0,QS18E.Read_Data.Quality_of_Teach,0,8)OTU(Port_Data.Port_Read.[Port])OTL(Local_Control.6);
   43: NOP();
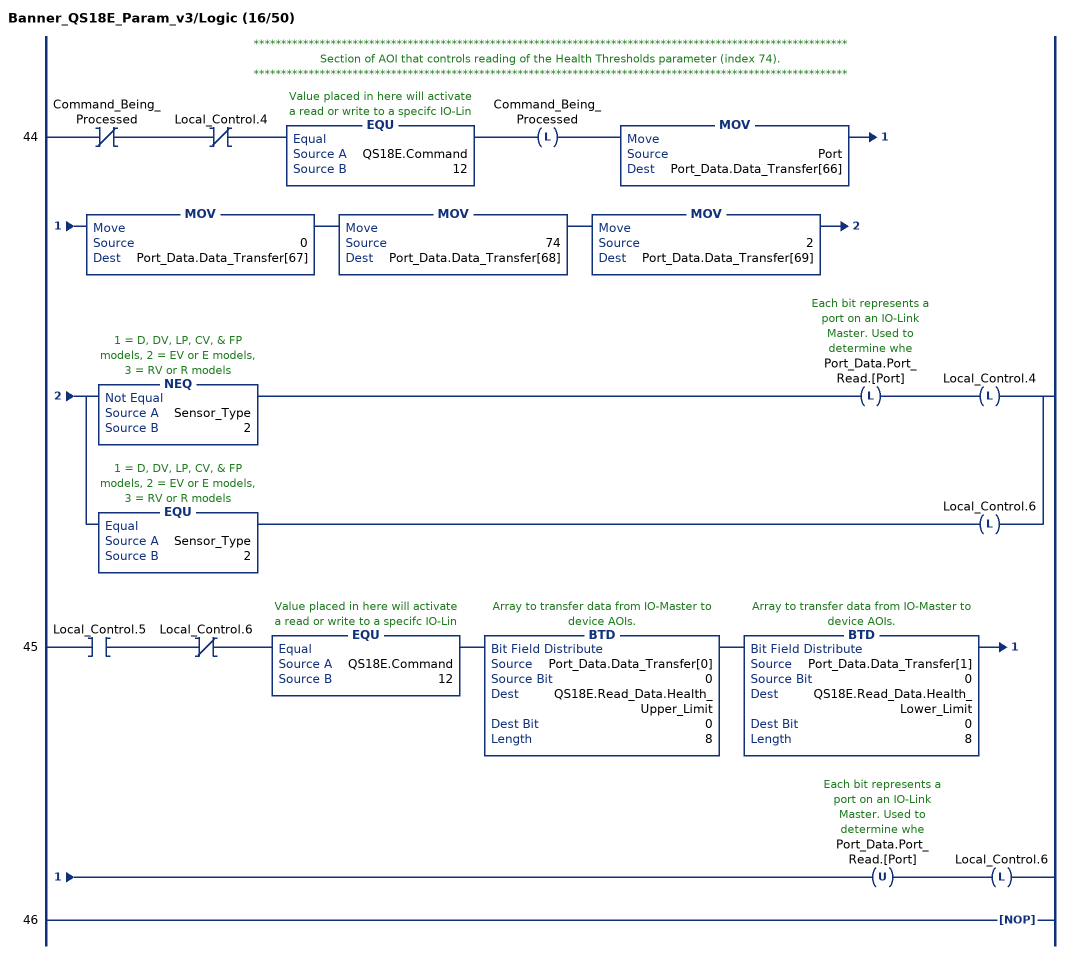
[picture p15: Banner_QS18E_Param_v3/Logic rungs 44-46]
   // ************************************************************************************************************
   // Section of AOI that controls reading of the Health Thresholds parameter (index 74).
   // ************************************************************************************************************
   44: XIO(Command_Being_Processed)XIO(Local_Control.4)EQU(QS18E.Command,12)OTL(Command_Being_Processed)MOV(Port,Port_Data.Data_Transfer[66])MOV(0,Port_Data.Data_Transfer[67])MOV(74,Port_Data.Data_Transfer[68])MOV(2,Port_Data.Data_Transfer[69])[NEQ(Sensor_Type,2) OTL(Port_Data.Port_Read.[Port]) OTL(Local_Control.4) ,EQU(Sensor_Type,2) OTL(Local_Control.6) ];
   45: XIC(Local_Control.5)XIO(Local_Control.6)EQU(QS18E.Command,12)BTD(Port_Data.Data_Transfer[0],0,QS18E.Read_Data.Health_Upper_Limit,0,8)BTD(Port_Data.Data_Transfer[1],0,QS18E.Read_Data.Health_Lower_Limit,0,8)OTU(Port_Data.Port_Read.[Port])OTL(Local_Control.6);
   46: NOP();
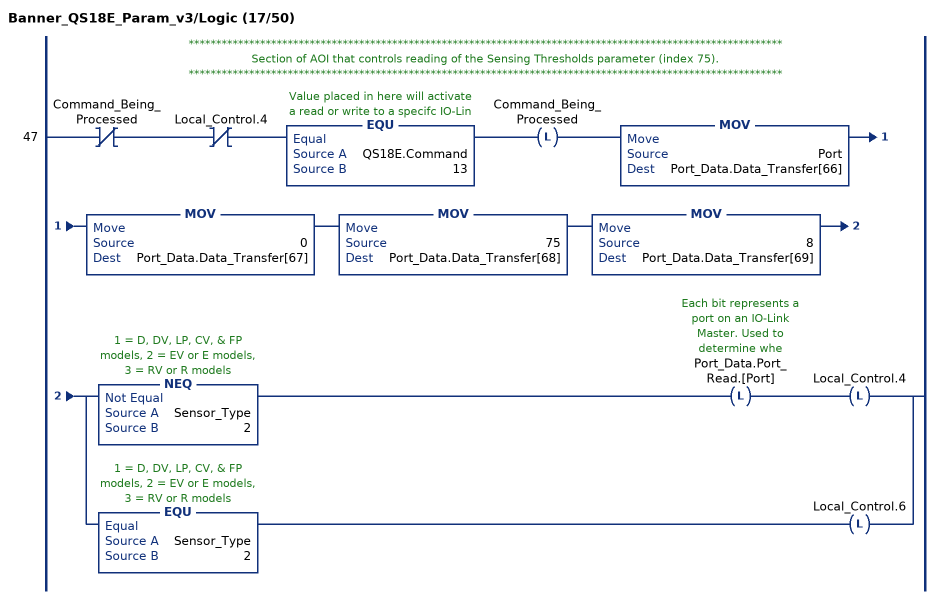
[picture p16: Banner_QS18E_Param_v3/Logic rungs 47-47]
   // ************************************************************************************************************
   // Section of AOI that controls reading of the Sensing Thresholds parameter (index 75).
   // ************************************************************************************************************
   47: XIO(Command_Being_Processed)XIO(Local_Control.4)EQU(QS18E.Command,13)OTL(Command_Being_Processed)MOV(Port,Port_Data.Data_Transfer[66])MOV(0,Port_Data.Data_Transfer[67])MOV(75,Port_Data.Data_Transfer[68])MOV(8,Port_Data.Data_Transfer[69])[NEQ(Sensor_Type,2) OTL(Port_Data.Port_Read.[Port]) OTL(Local_Control.4) ,EQU(Sensor_Type,2) OTL(Local_Control.6) ];
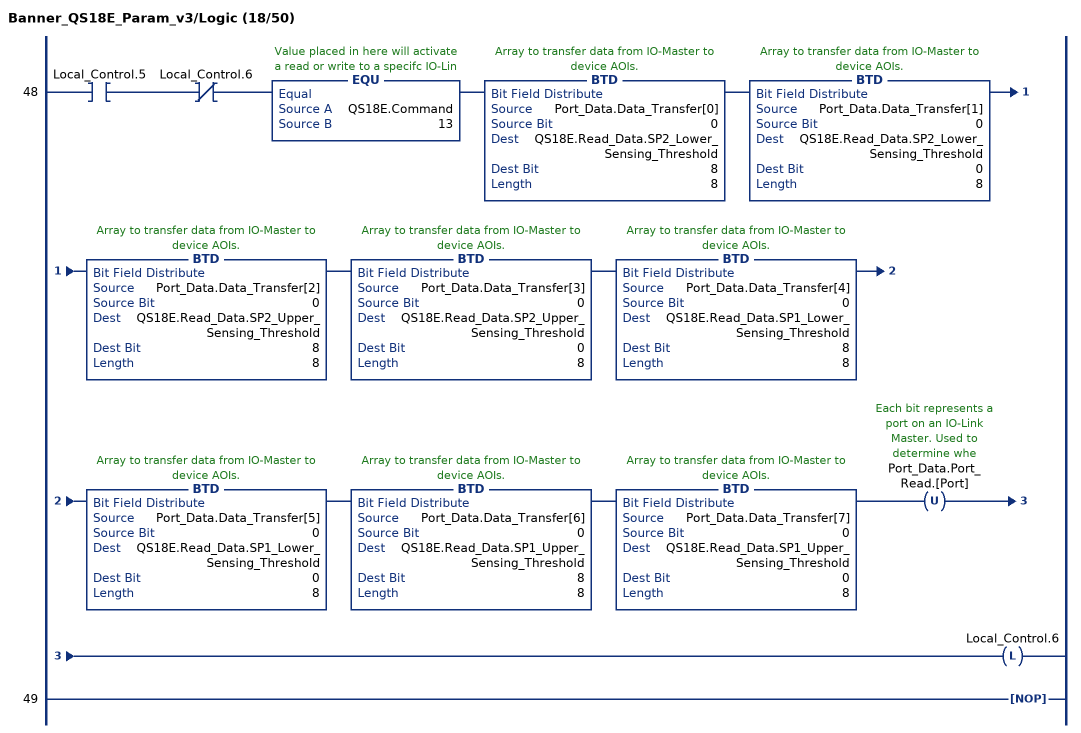
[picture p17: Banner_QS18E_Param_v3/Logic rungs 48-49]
   48: XIC(Local_Control.5)XIO(Local_Control.6)EQU(QS18E.Command,13)BTD(Port_Data.Data_Transfer[0],0,QS18E.Read_Data.SP2_Lower_Sensing_Threshold,8,8)BTD(Port_Data.Data_Transfer[1],0,QS18E.Read_Data.SP2_Lower_Sensing_Threshold,0,8)BTD(Port_Data.Data_Transfer[2],0,QS18E.Read_Data.SP2_Upper_Sensing_Threshold,8,8)BTD(Port_Data.Data_Transfer[3],0,QS18E.Read_Data.SP2_Upper_Sensing_Threshold,0,8)BTD(Port_Data.Data_Transfer[4],0,QS18E.Read_Data.SP1_Lower_Sensing_Threshold,8,8)BTD(Port_Data.Data_Transfer[5],0,QS18E.Read_Data.SP1_Lower_Sensing_Threshold,0,8)BTD(Port_Data.Data_Transfer[6],0,QS18E.Read_Data.SP1_Upper_Sensing_Threshold,8,8)BTD(Port_Data.Data_Transfer[7],0,QS18E.Read_Data.SP1_Upper_Sensing_Threshold,0,8)OTU(Port_Data.Port_Read.[Port])OTL(Local_Control.6);
   49: NOP();
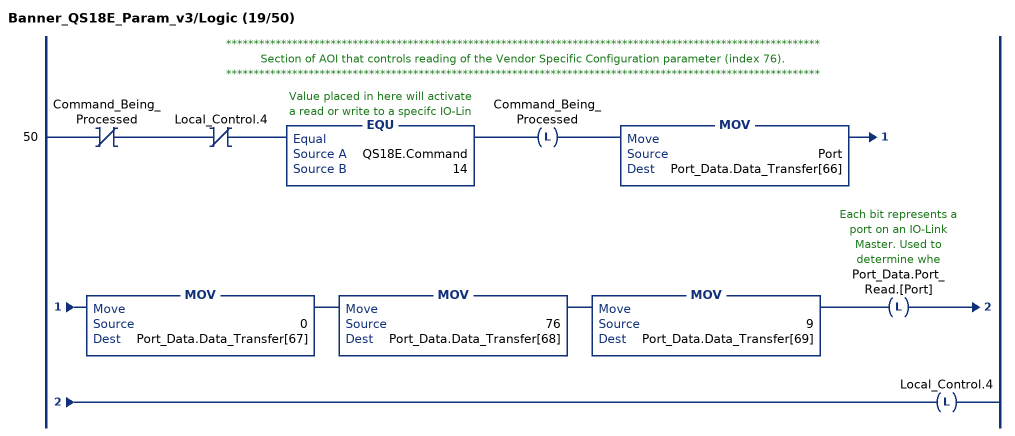
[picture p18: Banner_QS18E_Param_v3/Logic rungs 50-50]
   // ************************************************************************************************************
   // Section of AOI that controls reading of the Vendor Specific Configuration parameter (index 76).
   // ************************************************************************************************************
   50: XIO(Command_Being_Processed)XIO(Local_Control.4)EQU(QS18E.Command,14)OTL(Command_Being_Processed)MOV(Port,Port_Data.Data_Transfer[66])MOV(0,Port_Data.Data_Transfer[67])MOV(76,Port_Data.Data_Transfer[68])MOV(9,Port_Data.Data_Transfer[69])OTL(Port_Data.Port_Read.[Port])OTL(Local_Control.4);
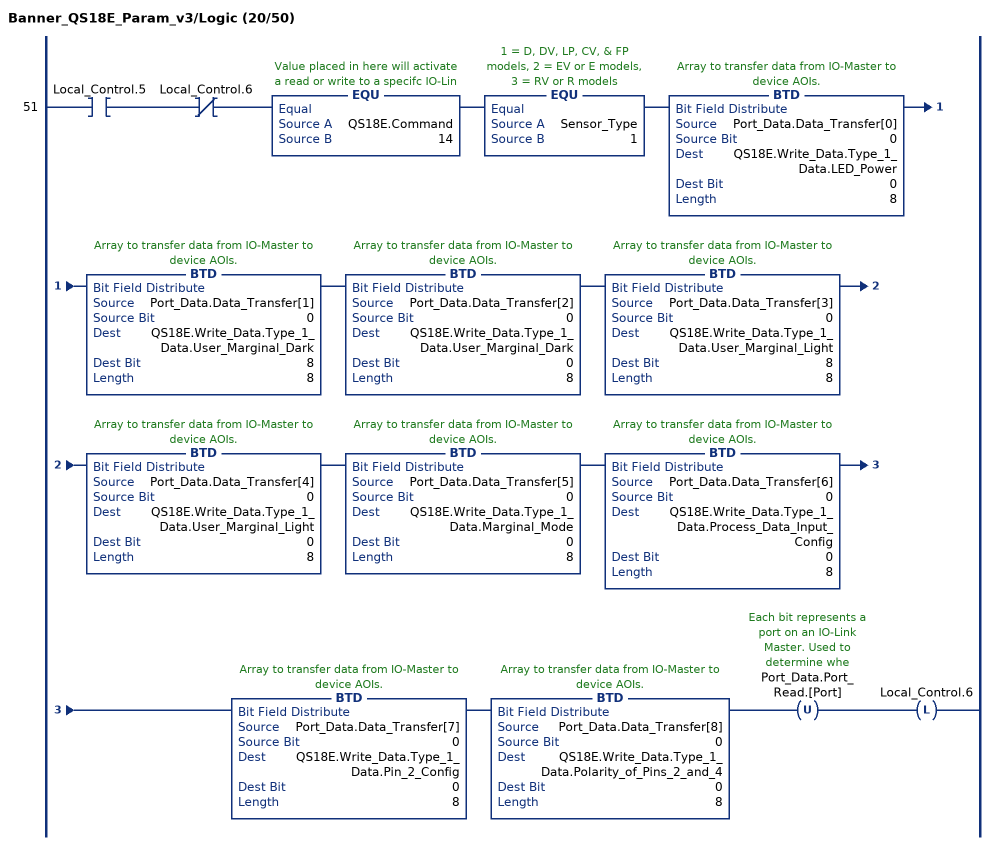
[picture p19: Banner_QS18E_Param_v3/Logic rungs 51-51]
   51: XIC(Local_Control.5)XIO(Local_Control.6)EQU(QS18E.Command,14)EQU(Sensor_Type,1)BTD(Port_Data.Data_Transfer[0],0,QS18E.Write_Data.Type_1_Data.LED_Power,0,8)BTD(Port_Data.Data_Transfer[1],0,QS18E.Write_Data.Type_1_Data.User_Marginal_Dark,8,8)BTD(Port_Data.Data_Transfer[2],0,QS18E.Write_Data.Type_1_Data.User_Marginal_Dark,0,8)BTD(Port_Data.Data_Transfer[3],0,QS18E.Write_Data.Type_1_Data.User_Marginal_Light,8,8)BTD(Port_Data.Data_Transfer[4],0,QS18E.Write_Data.Type_1_Data.User_Marginal_Light,0,8)BTD(Port_Data.Data_Transfer[5],0,QS18E.Write_Data.Type_1_Data.Marginal_Mode,0,8)BTD(Port_Data.Data_Transfer[6],0,QS18E.Write_Data.Type_1_Data.Process_Data_Input_Config,0,8)BTD(Port_Data.Data_Transfer[7],0,QS18E.Write_Data.Type_1_Data.Pin_2_Config,0,8)BTD(Port_Data.Data_Transfer[8],0,QS18E.Write_Data.Type_1_Data.Polarity_of_Pins_2_and_4,0,8)OTU(Port_Data.Port_Read.[Port])OTL(Local_Control.6);
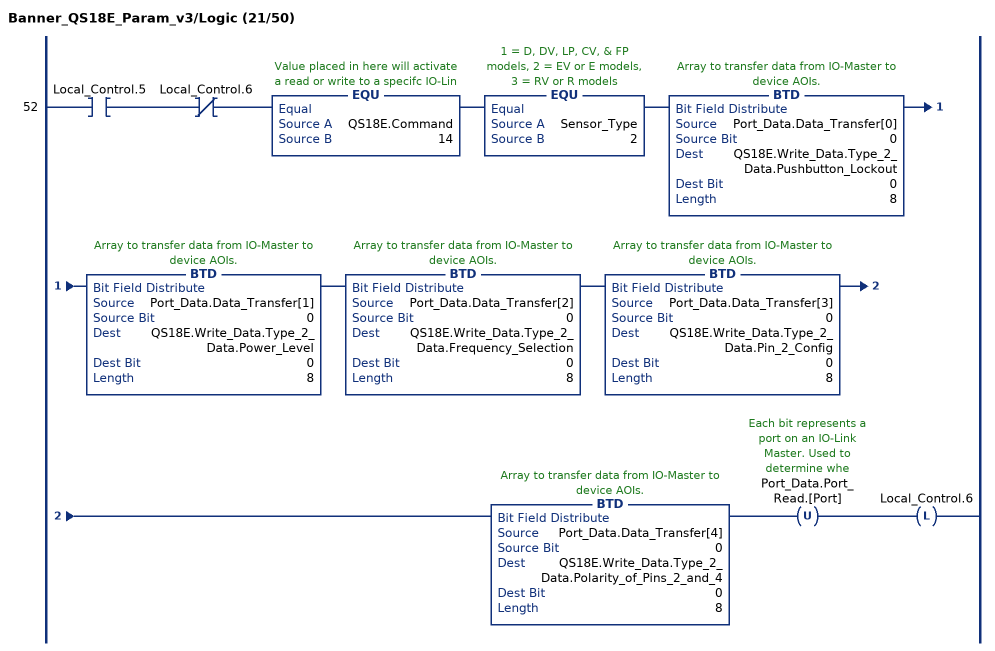
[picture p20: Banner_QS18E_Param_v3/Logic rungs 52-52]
   52: XIC(Local_Control.5)XIO(Local_Control.6)EQU(QS18E.Command,14)EQU(Sensor_Type,2)BTD(Port_Data.Data_Transfer[0],0,QS18E.Write_Data.Type_2_Data.Pushbutton_Lockout,0,8)BTD(Port_Data.Data_Transfer[1],0,QS18E.Write_Data.Type_2_Data.Power_Level,0,8)BTD(Port_Data.Data_Transfer[2],0,QS18E.Write_Data.Type_2_Data.Frequency_Selection,0,8)BTD(Port_Data.Data_Transfer[3],0,QS18E.Write_Data.Type_2_Data.Pin_2_Config,0,8)BTD(Port_Data.Data_Transfer[4],0,QS18E.Write_Data.Type_2_Data.Polarity_of_Pins_2_and_4,0,8)OTU(Port_Data.Port_Read.[Port])OTL(Local_Control.6);
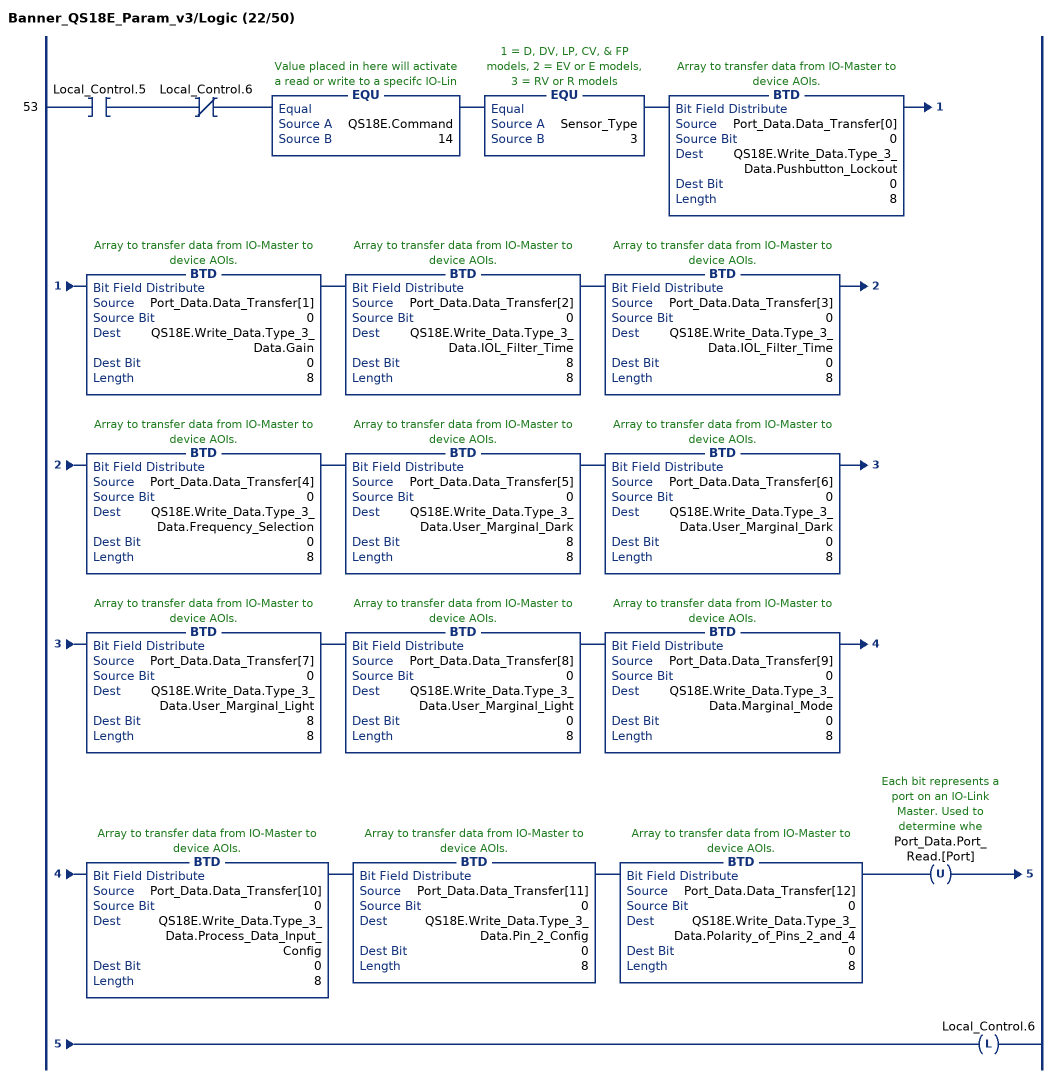
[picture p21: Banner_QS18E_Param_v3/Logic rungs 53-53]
   53: XIC(Local_Control.5)XIO(Local_Control.6)EQU(QS18E.Command,14)EQU(Sensor_Type,3)BTD(Port_Data.Data_Transfer[0],0,QS18E.Write_Data.Type_3_Data.Pushbutton_Lockout,0,8)BTD(Port_Data.Data_Transfer[1],0,QS18E.Write_Data.Type_3_Data.Gain,0,8)BTD(Port_Data.Data_Transfer[2],0,QS18E.Write_Data.Type_3_Data.IOL_Filter_Time,8,8)BTD(Port_Data.Data_Transfer[3],0,QS18E.Write_Data.Type_3_Data.IOL_Filter_Time,0,8)BTD(Port_Data.Data_Transfer[4],0,QS18E.Write_Data.Type_3_Data.Frequency_Selection,0,8)BTD(Port_Data.Data_Transfer[5],0,QS18E.Write_Data.Type_3_Data.User_Marginal_Dark,8,8)BTD(Port_Data.Data_Transfer[6],0,QS18E.Write_Data.Type_3_Data.User_Marginal_Dark,0,8)BTD(Port_Data.Data_Transfer[7],0,QS18E.Write_Data.Type_3_Data.User_Marginal_Light,8,8)BTD(Port_Data.Data_Transfer[8],0,QS18E.Write_Data.Type_3_Data.User_Marginal_Light,0,8)BTD(Port_Data.Data_Transfer[9],0,QS18E.Write_Data.Type_3_Data.Marginal_Mode,0,8)BTD(Port_Data.Data_Transfer[10],0,QS18E.Write_Data.Type_3_Data.Process_Data_Input_Config,0,8)BTD(Port_Data.Data_Transfer[11],0,QS18E.Write_Data.Type_3_Data.Pin_2_Config,0,8)BTD(Port_Data.Data_Transfer[12],0,QS18E.Write_Data.Type_3_Data.Polarity_of_Pins_2_and_4,0,8)OTU(Port_Data.Port_Read.[Port])OTL(Local_Control.6);
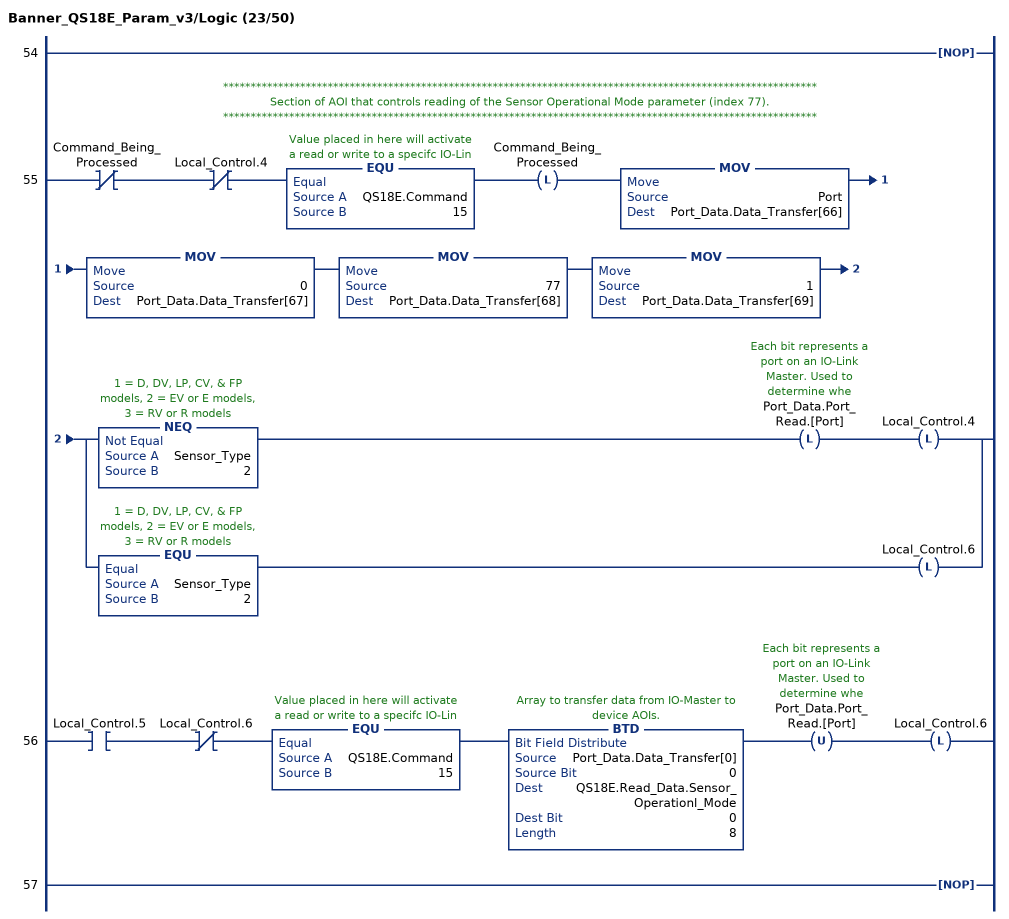
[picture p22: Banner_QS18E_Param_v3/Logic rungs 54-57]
   54: NOP();
   // ************************************************************************************************************
   // Section of AOI that controls reading of the Sensor Operational Mode parameter (index 77).
   // ************************************************************************************************************
   55: XIO(Command_Being_Processed)XIO(Local_Control.4)EQU(QS18E.Command,15)OTL(Command_Being_Processed)MOV(Port,Port_Data.Data_Transfer[66])MOV(0,Port_Data.Data_Transfer[67])MOV(77,Port_Data.Data_Transfer[68])MOV(1,Port_Data.Data_Transfer[69])[NEQ(Sensor_Type,2) OTL(Port_Data.Port_Read.[Port]) OTL(Local_Control.4) ,EQU(Sensor_Type,2) OTL(Local_Control.6) ];
   56: XIC(Local_Control.5)XIO(Local_Control.6)EQU(QS18E.Command,15)BTD(Port_Data.Data_Transfer[0],0,QS18E.Read_Data.Sensor_Operationl_Mode,0,8)OTU(Port_Data.Port_Read.[Port])OTL(Local_Control.6);
   57: NOP();
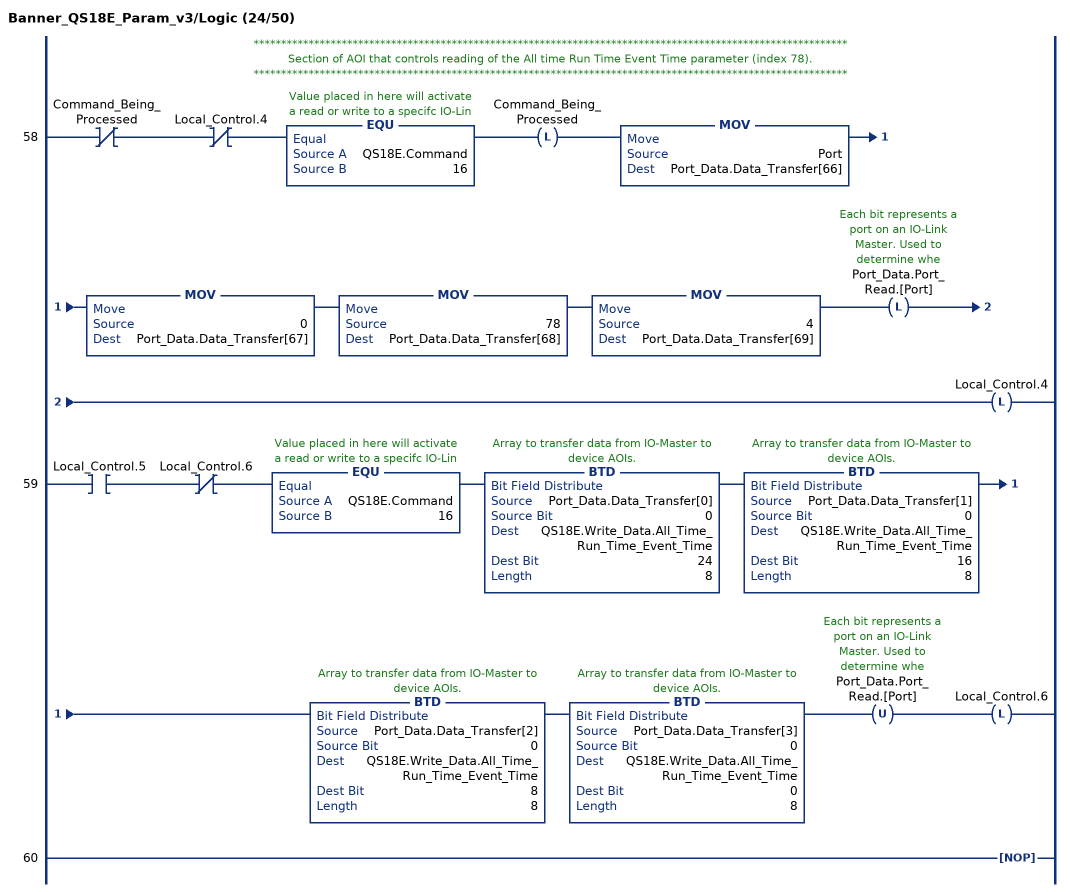
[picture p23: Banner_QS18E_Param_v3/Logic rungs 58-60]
   // ************************************************************************************************************
   // Section of AOI that controls reading of the All time Run Time Event Time parameter (index 78).
   // ************************************************************************************************************
   58: XIO(Command_Being_Processed)XIO(Local_Control.4)EQU(QS18E.Command,16)OTL(Command_Being_Processed)MOV(Port,Port_Data.Data_Transfer[66])MOV(0,Port_Data.Data_Transfer[67])MOV(78,Port_Data.Data_Transfer[68])MOV(4,Port_Data.Data_Transfer[69])OTL(Port_Data.Port_Read.[Port])OTL(Local_Control.4);
   59: XIC(Local_Control.5)XIO(Local_Control.6)EQU(QS18E.Command,16)BTD(Port_Data.Data_Transfer[0],0,QS18E.Write_Data.All_Time_Run_Time_Event_Time,24,8)BTD(Port_Data.Data_Transfer[1],0,QS18E.Write_Data.All_Time_Run_Time_Event_Time,16,8)BTD(Port_Data.Data_Transfer[2],0,QS18E.Write_Data.All_Time_Run_Time_Event_Time,8,8)BTD(Port_Data.Data_Transfer[3],0,QS18E.Write_Data.All_Time_Run_Time_Event_Time,0,8)OTU(Port_Data.Port_Read.[Port])OTL(Local_Control.6);
   60: NOP();
